(* Logix 5000 Program export KEP; software revision 30.00; part 13 of 15 *)
(* tags used below, declared in another part *)
   Ed25519_SIGN1 : Ed25519_SIGN;
   Ed25519_SIGN2 : Ed25519_SIGN;
   Ed25519_SIGN3 : Ed25519_SIGN;
   Ed25519_SIGN4 : Ed25519_SIGN;
   EdDSA_INTERNAL : EdDSA_INTERNAL[5];
   EdDSA_STATES : EdDSA_STATECTRL[15];
   InternalFlags : InternalFlags[5];
   InternalFlag_AllNodesUsingKsPrime : BOOL;
   InternalFlag_ALLOK : BOOL;
   InternalFlag_CreateNewKsPrime : BOOL;
   InternalFlag_KeyServerIdentityNo : BOOL;
   InternalFlag_KeyServerIdentityYes : BOOL;
   InternalFlag_KsEqualKsPrimeStatus : BOOL;
   InternalFlag_KsIDMatchesServer : BOOL;
   InternalFlag_KsPrimeAvail : BOOL;
   InternalFlag_KsPrimeIDMatchesServer : BOOL;
   InternalFlag_PowerOnCycle : BOOL;
   Internal_EdDSA_Msg : EdDSA_MSG;
   Internal_PriKeyPrefix : STRING;
   Internal_PriKeyScalar : STRING;
   Internal_PubKey : STRING;
   MyNodeNumber : DINT;
   ServerNode : INT;
   SignedMsgDest : INT;   // 0=None 1=Server 2=Client 3=All
   Temp_Processor_C1 : DINT[22];
   Temp_Processor_C10 : DINT[22];
   Temp_Processor_C2 : DINT[22];
   Temp_Processor_C3 : DINT[22];
   Temp_Processor_C4 : DINT[22];
   Temp_Processor_C5 : DINT[22];
   Temp_Processor_C6 : DINT[22];
   Temp_Processor_C7 : DINT[22];
   Temp_Processor_C8 : DINT[22];
   Temp_Processor_C9 : DINT[22];
   Temp_Processor_D1 : DINT[43];
   Temp_Processor_D2 : DINT[43];
   Temp_Processor_E1 : DINT[32];
   Temp_Processor_E2 : DINT[32];
   Temp_Processor_E3 : DINT[32];
   Temp_Processor_HASH : LINT[8];
   Temp_Processor_L : LINT[4];
   Temp_Processor_MSG : LINT[1600];
   Temp_Processor_P1 : POINT;
   Temp_Processor_P2 : POINT;
   Temp_Processor_P3 : POINT;
   Temp_Processor_P4 : POINT;
   Temp_Processor_S : STRING;
   T_INT1 : INT;
   WorkingNode : DINT;
   EdDSA_MSG_TO_NODE1 : EdDSA_MSG;
   EdDSA_MSG_TO_NODE2 : EdDSA_MSG;
   EdDSA_MSG_TO_NODE3 : EdDSA_MSG;
   EdDSA_MSG_TO_NODE4 : EdDSA_MSG;
   InternalFlag_KsID : LINT;
   InternalFlag_KsPrimeID : LINT;
   NODE : VMAC_DATA_INTERNAL[5];
(* KEP, continued *)

ROUTINE PROCESSOR_STATE4   (* ladder *)
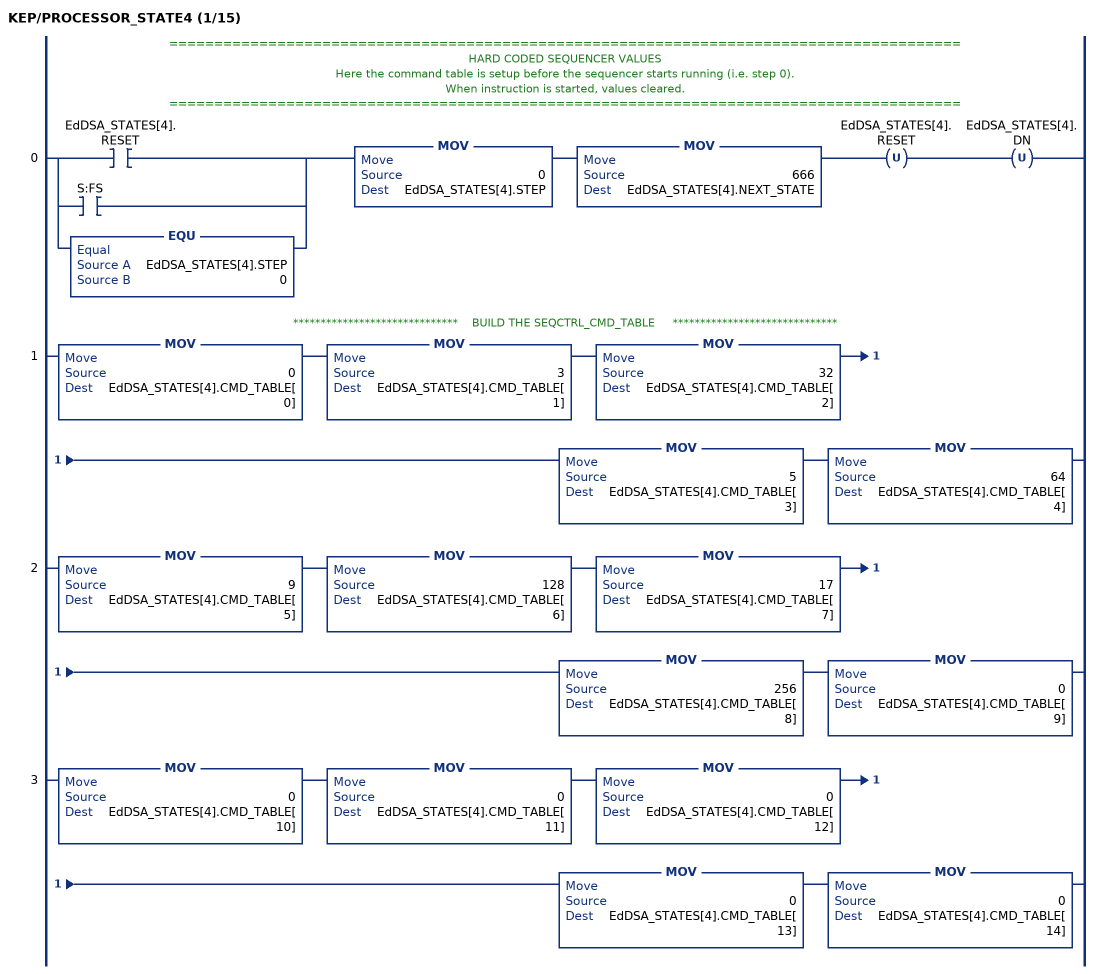
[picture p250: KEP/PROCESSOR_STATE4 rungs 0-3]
   // ========================================================================================
   // HARD CODED SEQUENCER VALUES
   // Here the command table is setup before the sequencer starts running (i.e. step 0).
   // When instruction is started, values cleared.
   // ========================================================================================
   0: [[XIC(EdDSA_STATES[4].RESET) ,XIC(S:FS) ] ,EQU(EdDSA_STATES[4].STEP,0) ]MOV(0,EdDSA_STATES[4].STEP)MOV(666,EdDSA_STATES[4].NEXT_STATE)OTU(EdDSA_STATES[4].RESET)OTU(EdDSA_STATES[4].DN);
   // ******************************    BUILD THE SEQCTRL_CMD_TABLE     ******************************
   1: MOV(0,EdDSA_STATES[4].CMD_TABLE[0])MOV(3,EdDSA_STATES[4].CMD_TABLE[1])MOV(32,EdDSA_STATES[4].CMD_TABLE[2])MOV(5,EdDSA_STATES[4].CMD_TABLE[3])MOV(64,EdDSA_STATES[4].CMD_TABLE[4]);
   2: MOV(9,EdDSA_STATES[4].CMD_TABLE[5])MOV(128,EdDSA_STATES[4].CMD_TABLE[6])MOV(17,EdDSA_STATES[4].CMD_TABLE[7])MOV(256,EdDSA_STATES[4].CMD_TABLE[8])MOV(0,EdDSA_STATES[4].CMD_TABLE[9]);
   3: MOV(0,EdDSA_STATES[4].CMD_TABLE[10])MOV(0,EdDSA_STATES[4].CMD_TABLE[11])MOV(0,EdDSA_STATES[4].CMD_TABLE[12])MOV(0,EdDSA_STATES[4].CMD_TABLE[13])MOV(0,EdDSA_STATES[4].CMD_TABLE[14]);
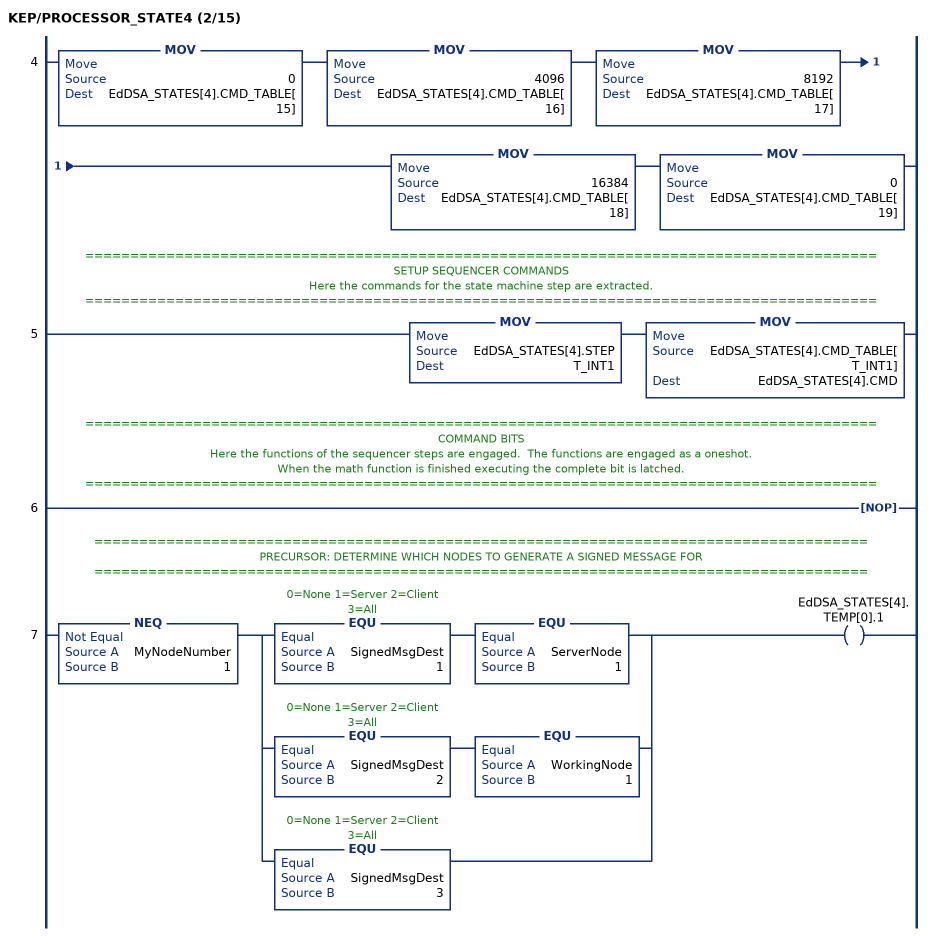
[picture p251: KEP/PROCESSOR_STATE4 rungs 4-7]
   4: MOV(0,EdDSA_STATES[4].CMD_TABLE[15])MOV(4096,EdDSA_STATES[4].CMD_TABLE[16])MOV(8192,EdDSA_STATES[4].CMD_TABLE[17])MOV(16384,EdDSA_STATES[4].CMD_TABLE[18])MOV(0,EdDSA_STATES[4].CMD_TABLE[19]);
   // ========================================================================================
   // SETUP SEQUENCER COMMANDS
   // Here the commands for the state machine step are extracted.
   // ========================================================================================
   5: MOV(EdDSA_STATES[4].STEP,T_INT1)MOV(EdDSA_STATES[4].CMD_TABLE[T_INT1],EdDSA_STATES[4].CMD);
   // ========================================================================================
   // COMMAND BITS
   // Here the functions of the sequencer steps are engaged.  The functions are engaged as a oneshot.
   // When the math function is finished executing the complete bit is latched.
   // ========================================================================================
   6: NOP();
   // ======================================================================================
   // PRECURSOR: DETERMINE WHICH NODES TO GENERATE A SIGNED MESSAGE FOR
   // ======================================================================================
   7: NEQ(MyNodeNumber,1)[EQU(SignedMsgDest,1) EQU(ServerNode,1) ,EQU(SignedMsgDest,2) EQU(WorkingNode,1) ,EQU(SignedMsgDest,3) ]OTE(EdDSA_STATES[4].TEMP[0].1);
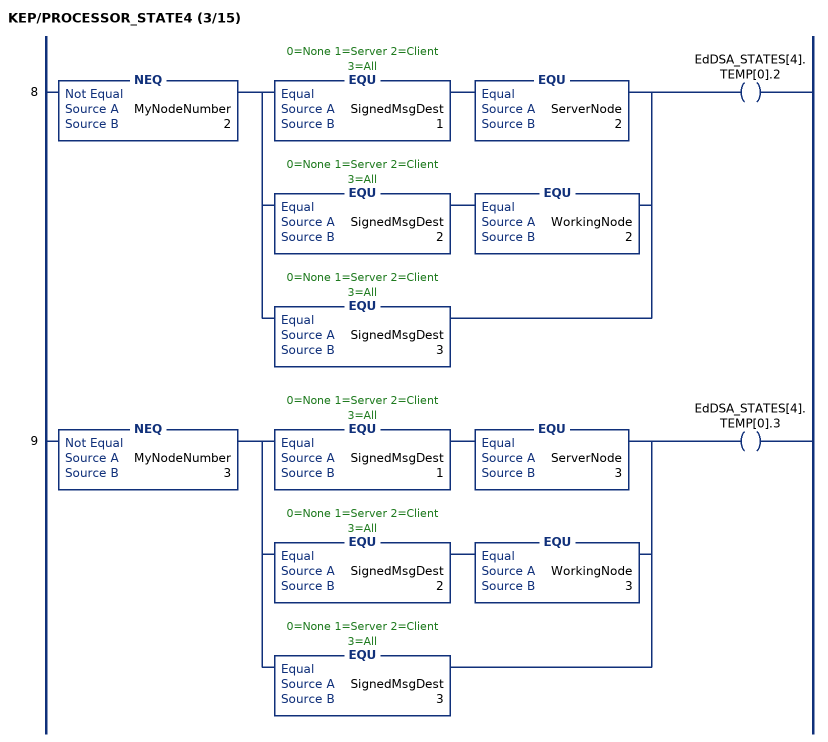
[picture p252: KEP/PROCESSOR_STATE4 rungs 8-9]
   8: NEQ(MyNodeNumber,2)[EQU(SignedMsgDest,1) EQU(ServerNode,2) ,EQU(SignedMsgDest,2) EQU(WorkingNode,2) ,EQU(SignedMsgDest,3) ]OTE(EdDSA_STATES[4].TEMP[0].2);
   9: NEQ(MyNodeNumber,3)[EQU(SignedMsgDest,1) EQU(ServerNode,3) ,EQU(SignedMsgDest,2) EQU(WorkingNode,3) ,EQU(SignedMsgDest,3) ]OTE(EdDSA_STATES[4].TEMP[0].3);
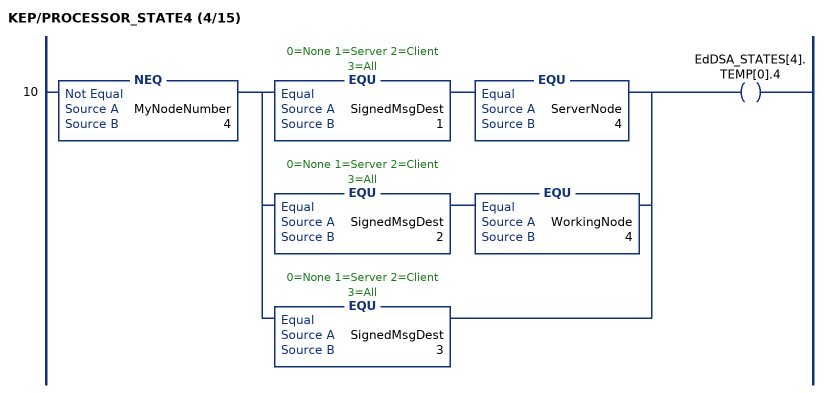
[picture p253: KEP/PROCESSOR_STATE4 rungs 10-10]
   10: NEQ(MyNodeNumber,4)[EQU(SignedMsgDest,1) EQU(ServerNode,4) ,EQU(SignedMsgDest,2) EQU(WorkingNode,4) ,EQU(SignedMsgDest,3) ]OTE(EdDSA_STATES[4].TEMP[0].4);
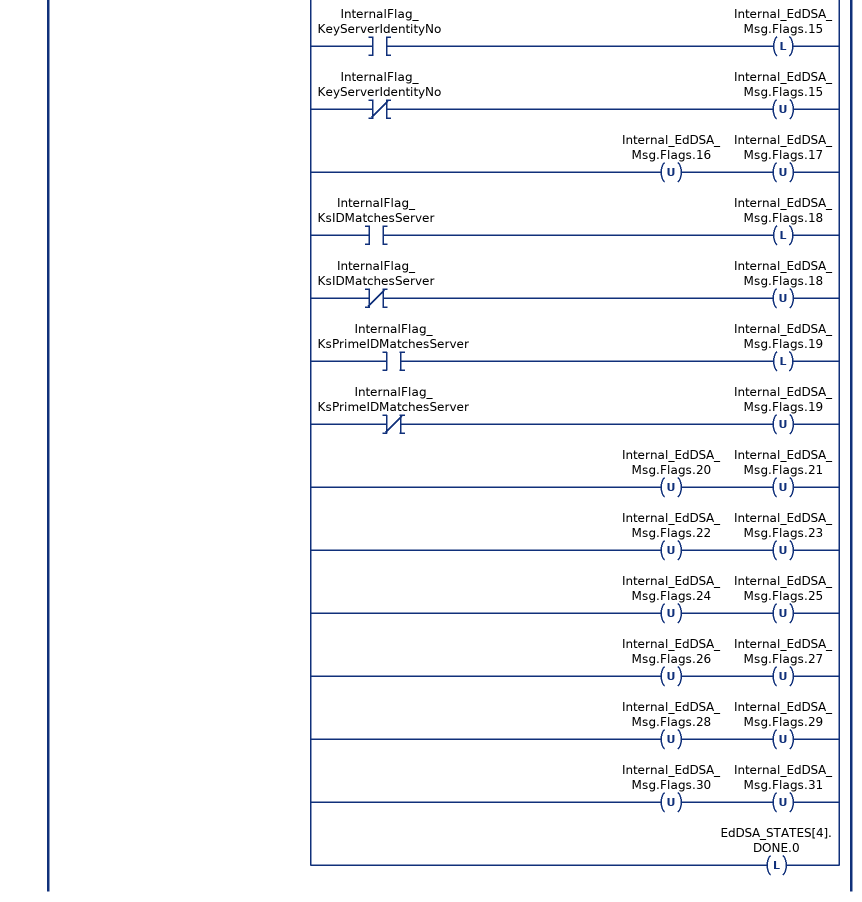
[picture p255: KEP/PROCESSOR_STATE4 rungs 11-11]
   // ======================================================================================
   // PART 0: MAP KEY IDENTITY AND COMMON FLAGS TO INTERNAL EdDSA MESSAGE
   // ======================================================================================
   11: XIC(EdDSA_STATES[4].CMD.0)XIO(EdDSA_STATES[4].DONE.0)[COP(InternalFlag_KsID,Internal_EdDSA_Msg.KsID,1) COP(InternalFlag_KsPrimeID,Internal_EdDSA_Msg.KsPrimeID,1) ,[XIC(InternalFlag_ALLOK) OTL(Internal_EdDSA_Msg.Flags.0) ,XIO(InternalFlag_ALLOK) OTU(Internal_EdDSA_Msg.Flags.0) ] ,OTU(Internal_EdDSA_Msg.Flags.1) OTU(Internal_EdDSA_Msg.Flags.2) ,OTU(Internal_EdDSA_Msg.Flags.3) OTU(Internal_EdDSA_Msg.Flags.4) ,OTU(Internal_EdDSA_Msg.Flags.5) OTU(Internal_EdDSA_Msg.Flags.6) ,[XIC(InternalFlag_KsPrimeAvail) OTL(Internal_EdDSA_Msg.Flags.9) ,XIO(InternalFlag_KsPrimeAvail) OTU(Internal_EdDSA_Msg.Flags.9) ] ,OTU(Internal_EdDSA_Msg.Flags.10) OTU(Internal_EdDSA_Msg.Flags.11) ,[XIC(InternalFlag_KsEqualKsPrimeStatus) OTL(Internal_EdDSA_Msg.Flags.12) ,XIO(InternalFlag_KsEqualKsPrimeStatus) OTU(Internal_EdDSA_Msg.Flags.12) ] ,OTU(Internal_EdDSA_Msg.Flags.13) ,[XIC(InternalFlag_KeyServerIdentityYes) OTL(Internal_EdDSA_Msg.Flags.14) ,XIO(InternalFlag_KeyServerIdentityYes) OTU(Internal_EdDSA_Msg.Flags.14) ] ,[XIC(InternalFlag_KeyServerIdentityNo) OTL(Internal_EdDSA_Msg.Flags.15) ,XIO(InternalFlag_KeyServerIdentityNo) OTU(Internal_EdDSA_Msg.Flags.15) ] ,OTU(Internal_EdDSA_Msg.Flags.16) OTU(Internal_EdDSA_Msg.Flags.17) ,[XIC(InternalFlag_KsIDMatchesServer) OTL(Internal_EdDSA_Msg.Flags.18) ,XIO(InternalFlag_KsIDMatchesServer) OTU(Internal_EdDSA_Msg.Flags.18) ] ,[XIC(InternalFlag_KsPrimeIDMatchesServer) OTL(Internal_EdDSA_Msg.Flags.19) ,XIO(InternalFlag_KsPrimeIDMatchesServer) OTU(Internal_EdDSA_Msg.Flags.19) ] ,OTU(Internal_EdDSA_Msg.Flags.20) OTU(Internal_EdDSA_Msg.Flags.21) ,OTU(Internal_EdDSA_Msg.Flags.22) OTU(Internal_EdDSA_Msg.Flags.23) ,OTU(Internal_EdDSA_Msg.Flags.24) OTU(Internal_EdDSA_Msg.Flags.25) ,OTU(Internal_EdDSA_Msg.Flags.26) OTU(Internal_EdDSA_Msg.Flags.27) ,OTU(Internal_EdDSA_Msg.Flags.28) OTU(Internal_EdDSA_Msg.Flags.29) ,OTU(Internal_EdDSA_Msg.Flags.30) OTU(Internal_EdDSA_Msg.Flags.31) ,OTL(EdDSA_STATES[4].DONE.0) ];
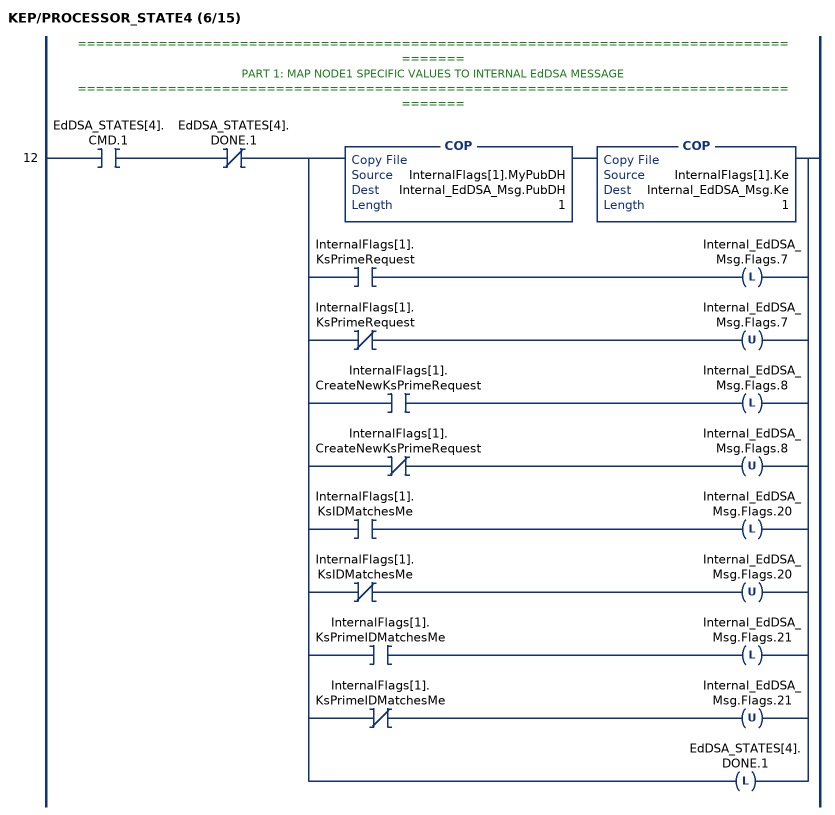
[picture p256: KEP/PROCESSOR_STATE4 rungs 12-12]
   // ======================================================================================
   // PART 1: MAP NODE1 SPECIFIC VALUES TO INTERNAL EdDSA MESSAGE
   // ======================================================================================
   12: XIC(EdDSA_STATES[4].CMD.1)XIO(EdDSA_STATES[4].DONE.1)[COP(InternalFlags[1].MyPubDH,Internal_EdDSA_Msg.PubDH,1) COP(InternalFlags[1].Ke,Internal_EdDSA_Msg.Ke,1) ,[XIC(InternalFlags[1].KsPrimeRequest) OTL(Internal_EdDSA_Msg.Flags.7) ,XIO(InternalFlags[1].KsPrimeRequest) OTU(Internal_EdDSA_Msg.Flags.7) ] ,[XIC(InternalFlags[1].CreateNewKsPrimeRequest) OTL(Internal_EdDSA_Msg.Flags.8) ,XIO(InternalFlags[1].CreateNewKsPrimeRequest) OTU(Internal_EdDSA_Msg.Flags.8) ] ,[XIC(InternalFlags[1].KsIDMatchesMe) OTL(Internal_EdDSA_Msg.Flags.20) ,XIO(InternalFlags[1].KsIDMatchesMe) OTU(Internal_EdDSA_Msg.Flags.20) ] ,[XIC(InternalFlags[1].KsPrimeIDMatchesMe) OTL(Internal_EdDSA_Msg.Flags.21) ,XIO(InternalFlags[1].KsPrimeIDMatchesMe) OTU(Internal_EdDSA_Msg.Flags.21) ] ,OTL(EdDSA_STATES[4].DONE.1) ];
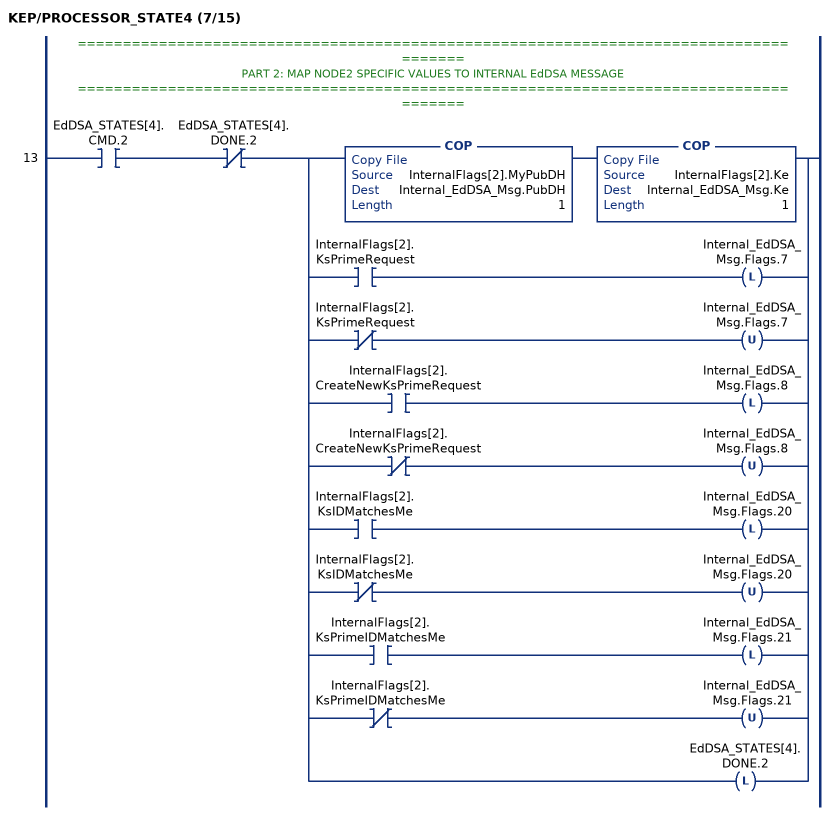
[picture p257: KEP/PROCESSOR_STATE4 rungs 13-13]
   // ======================================================================================
   // PART 2: MAP NODE2 SPECIFIC VALUES TO INTERNAL EdDSA MESSAGE
   // ======================================================================================
   13: XIC(EdDSA_STATES[4].CMD.2)XIO(EdDSA_STATES[4].DONE.2)[COP(InternalFlags[2].MyPubDH,Internal_EdDSA_Msg.PubDH,1) COP(InternalFlags[2].Ke,Internal_EdDSA_Msg.Ke,1) ,[XIC(InternalFlags[2].KsPrimeRequest) OTL(Internal_EdDSA_Msg.Flags.7) ,XIO(InternalFlags[2].KsPrimeRequest) OTU(Internal_EdDSA_Msg.Flags.7) ] ,[XIC(InternalFlags[2].CreateNewKsPrimeRequest) OTL(Internal_EdDSA_Msg.Flags.8) ,XIO(InternalFlags[2].CreateNewKsPrimeRequest) OTU(Internal_EdDSA_Msg.Flags.8) ] ,[XIC(InternalFlags[2].KsIDMatchesMe) OTL(Internal_EdDSA_Msg.Flags.20) ,XIO(InternalFlags[2].KsIDMatchesMe) OTU(Internal_EdDSA_Msg.Flags.20) ] ,[XIC(InternalFlags[2].KsPrimeIDMatchesMe) OTL(Internal_EdDSA_Msg.Flags.21) ,XIO(InternalFlags[2].KsPrimeIDMatchesMe) OTU(Internal_EdDSA_Msg.Flags.21) ] ,OTL(EdDSA_STATES[4].DONE.2) ];
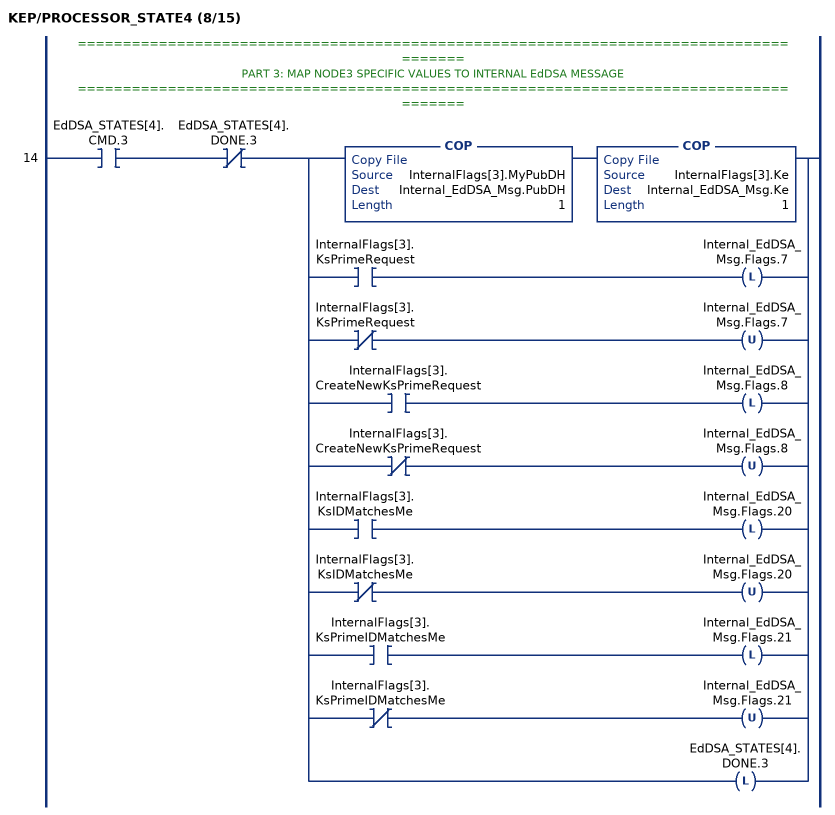
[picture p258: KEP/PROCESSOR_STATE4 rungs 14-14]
   // ======================================================================================
   // PART 3: MAP NODE3 SPECIFIC VALUES TO INTERNAL EdDSA MESSAGE
   // ======================================================================================
   14: XIC(EdDSA_STATES[4].CMD.3)XIO(EdDSA_STATES[4].DONE.3)[COP(InternalFlags[3].MyPubDH,Internal_EdDSA_Msg.PubDH,1) COP(InternalFlags[3].Ke,Internal_EdDSA_Msg.Ke,1) ,[XIC(InternalFlags[3].KsPrimeRequest) OTL(Internal_EdDSA_Msg.Flags.7) ,XIO(InternalFlags[3].KsPrimeRequest) OTU(Internal_EdDSA_Msg.Flags.7) ] ,[XIC(InternalFlags[3].CreateNewKsPrimeRequest) OTL(Internal_EdDSA_Msg.Flags.8) ,XIO(InternalFlags[3].CreateNewKsPrimeRequest) OTU(Internal_EdDSA_Msg.Flags.8) ] ,[XIC(InternalFlags[3].KsIDMatchesMe) OTL(Internal_EdDSA_Msg.Flags.20) ,XIO(InternalFlags[3].KsIDMatchesMe) OTU(Internal_EdDSA_Msg.Flags.20) ] ,[XIC(InternalFlags[3].KsPrimeIDMatchesMe) OTL(Internal_EdDSA_Msg.Flags.21) ,XIO(InternalFlags[3].KsPrimeIDMatchesMe) OTU(Internal_EdDSA_Msg.Flags.21) ] ,OTL(EdDSA_STATES[4].DONE.3) ];
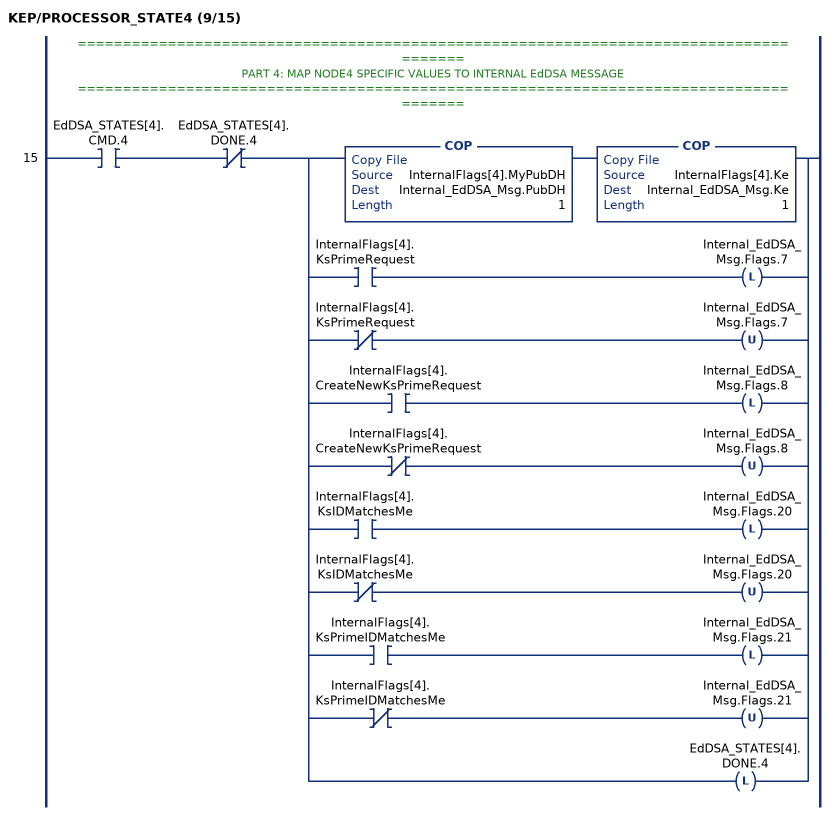
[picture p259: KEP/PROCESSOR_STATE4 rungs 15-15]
   // ======================================================================================
   // PART 4: MAP NODE4 SPECIFIC VALUES TO INTERNAL EdDSA MESSAGE
   // ======================================================================================
   15: XIC(EdDSA_STATES[4].CMD.4)XIO(EdDSA_STATES[4].DONE.4)[COP(InternalFlags[4].MyPubDH,Internal_EdDSA_Msg.PubDH,1) COP(InternalFlags[4].Ke,Internal_EdDSA_Msg.Ke,1) ,[XIC(InternalFlags[4].KsPrimeRequest) OTL(Internal_EdDSA_Msg.Flags.7) ,XIO(InternalFlags[4].KsPrimeRequest) OTU(Internal_EdDSA_Msg.Flags.7) ] ,[XIC(InternalFlags[4].CreateNewKsPrimeRequest) OTL(Internal_EdDSA_Msg.Flags.8) ,XIO(InternalFlags[4].CreateNewKsPrimeRequest) OTU(Internal_EdDSA_Msg.Flags.8) ] ,[XIC(InternalFlags[4].KsIDMatchesMe) OTL(Internal_EdDSA_Msg.Flags.20) ,XIO(InternalFlags[4].KsIDMatchesMe) OTU(Internal_EdDSA_Msg.Flags.20) ] ,[XIC(InternalFlags[4].KsPrimeIDMatchesMe) OTL(Internal_EdDSA_Msg.Flags.21) ,XIO(InternalFlags[4].KsPrimeIDMatchesMe) OTU(Internal_EdDSA_Msg.Flags.21) ] ,OTL(EdDSA_STATES[4].DONE.4) ];
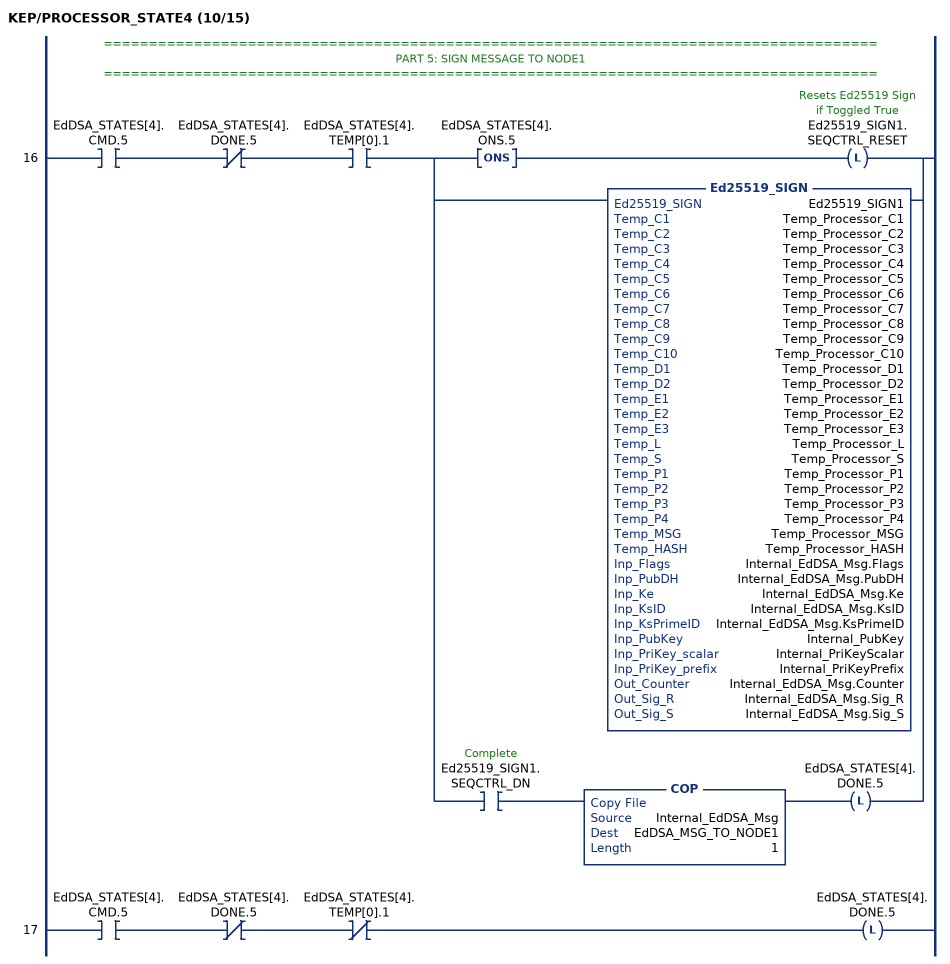
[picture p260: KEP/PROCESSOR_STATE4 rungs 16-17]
   // ======================================================================================
   // PART 5: SIGN MESSAGE TO NODE1
   // ======================================================================================
   16: XIC(EdDSA_STATES[4].CMD.5)XIO(EdDSA_STATES[4].DONE.5)XIC(EdDSA_STATES[4].TEMP[0].1)[ONS(EdDSA_STATES[4].ONS.5) OTL(Ed25519_SIGN1.SEQCTRL_RESET) ,Ed25519_SIGN(Ed25519_SIGN1,Temp_Processor_C1,Temp_Processor_C2,Temp_Processor_C3,Temp_Processor_C4,Temp_Processor_C5,Temp_Processor_C6,Temp_Processor_C7,Temp_Processor_C8,Temp_Processor_C9,Temp_Processor_C10,Temp_Processor_D1,Temp_Processor_D2,Temp_Processor_E1,Temp_Processor_E2,Temp_Processor_E3,Temp_Processor_L,Temp_Processor_S,Temp_Processor_P1,Temp_Processor_P2,Temp_Processor_P3,Temp_Processor_P4,Temp_Processor_MSG,Temp_Processor_HASH,Internal_EdDSA_Msg.Flags,Internal_EdDSA_Msg.PubDH,Internal_EdDSA_Msg.Ke,Internal_EdDSA_Msg.KsID,Internal_EdDSA_Msg.KsPrimeID,Internal_PubKey,Internal_PriKeyScalar,Internal_PriKeyPrefix,Internal_EdDSA_Msg.Counter,Internal_EdDSA_Msg.Sig_R,Internal_EdDSA_Msg.Sig_S) ,XIC(Ed25519_SIGN1.SEQCTRL_DN) COP(Internal_EdDSA_Msg,EdDSA_MSG_TO_NODE1,1) OTL(EdDSA_STATES[4].DONE.5) ];
   17: XIC(EdDSA_STATES[4].CMD.5)XIO(EdDSA_STATES[4].DONE.5)XIO(EdDSA_STATES[4].TEMP[0].1)OTL(EdDSA_STATES[4].DONE.5);
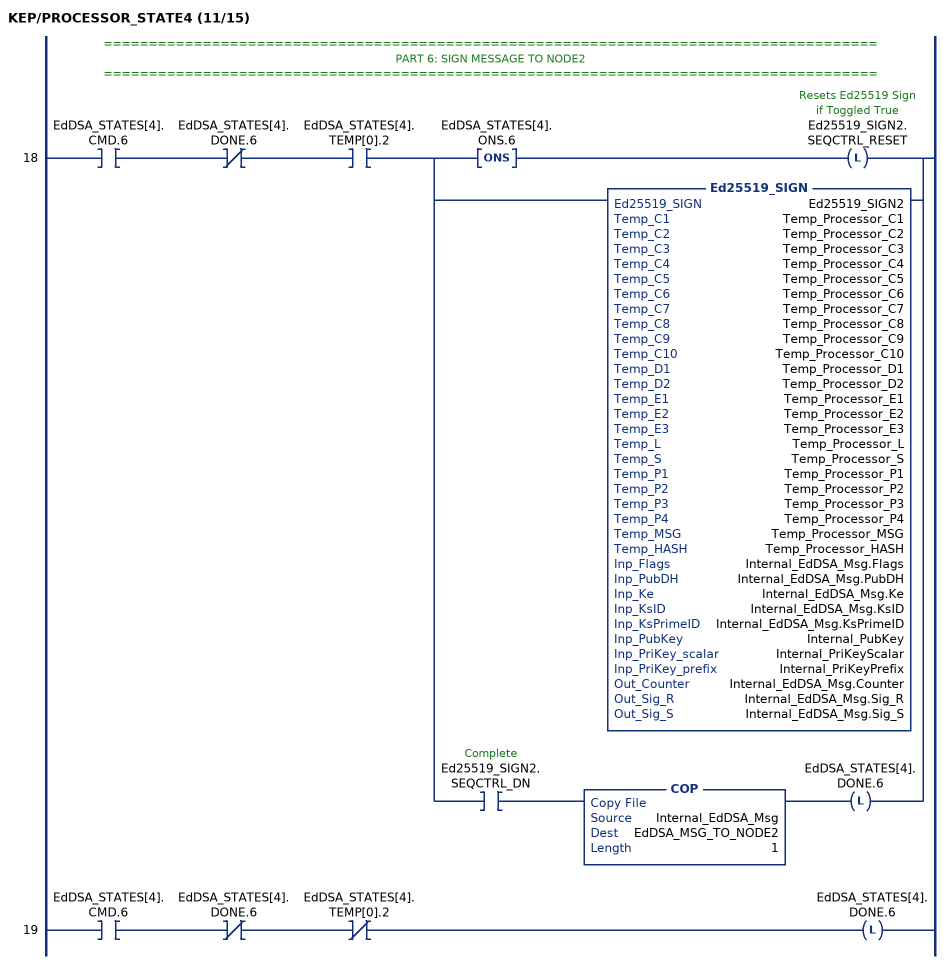
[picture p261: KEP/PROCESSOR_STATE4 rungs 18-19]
   // ======================================================================================
   // PART 6: SIGN MESSAGE TO NODE2
   // ======================================================================================
   18: XIC(EdDSA_STATES[4].CMD.6)XIO(EdDSA_STATES[4].DONE.6)XIC(EdDSA_STATES[4].TEMP[0].2)[ONS(EdDSA_STATES[4].ONS.6) OTL(Ed25519_SIGN2.SEQCTRL_RESET) ,Ed25519_SIGN(Ed25519_SIGN2,Temp_Processor_C1,Temp_Processor_C2,Temp_Processor_C3,Temp_Processor_C4,Temp_Processor_C5,Temp_Processor_C6,Temp_Processor_C7,Temp_Processor_C8,Temp_Processor_C9,Temp_Processor_C10,Temp_Processor_D1,Temp_Processor_D2,Temp_Processor_E1,Temp_Processor_E2,Temp_Processor_E3,Temp_Processor_L,Temp_Processor_S,Temp_Processor_P1,Temp_Processor_P2,Temp_Processor_P3,Temp_Processor_P4,Temp_Processor_MSG,Temp_Processor_HASH,Internal_EdDSA_Msg.Flags,Internal_EdDSA_Msg.PubDH,Internal_EdDSA_Msg.Ke,Internal_EdDSA_Msg.KsID,Internal_EdDSA_Msg.KsPrimeID,Internal_PubKey,Internal_PriKeyScalar,Internal_PriKeyPrefix,Internal_EdDSA_Msg.Counter,Internal_EdDSA_Msg.Sig_R,Internal_EdDSA_Msg.Sig_S) ,XIC(Ed25519_SIGN2.SEQCTRL_DN) COP(Internal_EdDSA_Msg,EdDSA_MSG_TO_NODE2,1) OTL(EdDSA_STATES[4].DONE.6) ];
   19: XIC(EdDSA_STATES[4].CMD.6)XIO(EdDSA_STATES[4].DONE.6)XIO(EdDSA_STATES[4].TEMP[0].2)OTL(EdDSA_STATES[4].DONE.6);
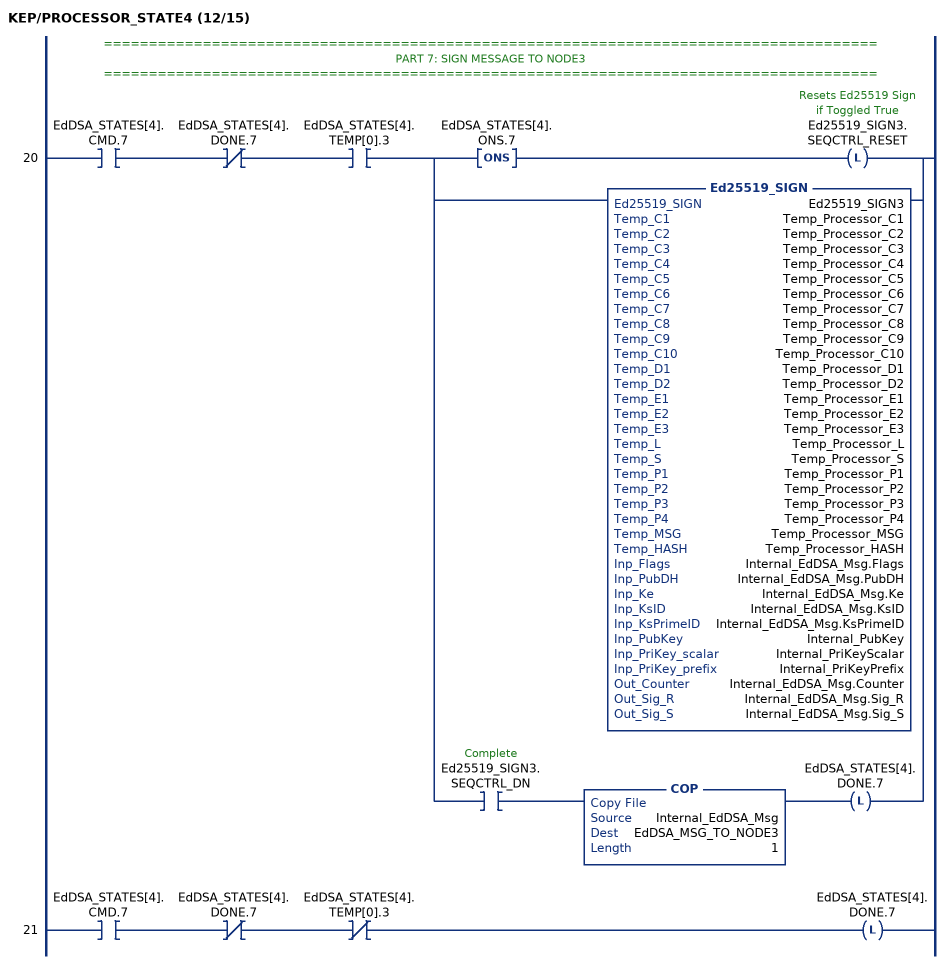
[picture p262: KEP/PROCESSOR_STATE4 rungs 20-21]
   // ======================================================================================
   // PART 7: SIGN MESSAGE TO NODE3
   // ======================================================================================
   20: XIC(EdDSA_STATES[4].CMD.7)XIO(EdDSA_STATES[4].DONE.7)XIC(EdDSA_STATES[4].TEMP[0].3)[ONS(EdDSA_STATES[4].ONS.7) OTL(Ed25519_SIGN3.SEQCTRL_RESET) ,Ed25519_SIGN(Ed25519_SIGN3,Temp_Processor_C1,Temp_Processor_C2,Temp_Processor_C3,Temp_Processor_C4,Temp_Processor_C5,Temp_Processor_C6,Temp_Processor_C7,Temp_Processor_C8,Temp_Processor_C9,Temp_Processor_C10,Temp_Processor_D1,Temp_Processor_D2,Temp_Processor_E1,Temp_Processor_E2,Temp_Processor_E3,Temp_Processor_L,Temp_Processor_S,Temp_Processor_P1,Temp_Processor_P2,Temp_Processor_P3,Temp_Processor_P4,Temp_Processor_MSG,Temp_Processor_HASH,Internal_EdDSA_Msg.Flags,Internal_EdDSA_Msg.PubDH,Internal_EdDSA_Msg.Ke,Internal_EdDSA_Msg.KsID,Internal_EdDSA_Msg.KsPrimeID,Internal_PubKey,Internal_PriKeyScalar,Internal_PriKeyPrefix,Internal_EdDSA_Msg.Counter,Internal_EdDSA_Msg.Sig_R,Internal_EdDSA_Msg.Sig_S) ,XIC(Ed25519_SIGN3.SEQCTRL_DN) COP(Internal_EdDSA_Msg,EdDSA_MSG_TO_NODE3,1) OTL(EdDSA_STATES[4].DONE.7) ];
   21: XIC(EdDSA_STATES[4].CMD.7)XIO(EdDSA_STATES[4].DONE.7)XIO(EdDSA_STATES[4].TEMP[0].3)OTL(EdDSA_STATES[4].DONE.7);
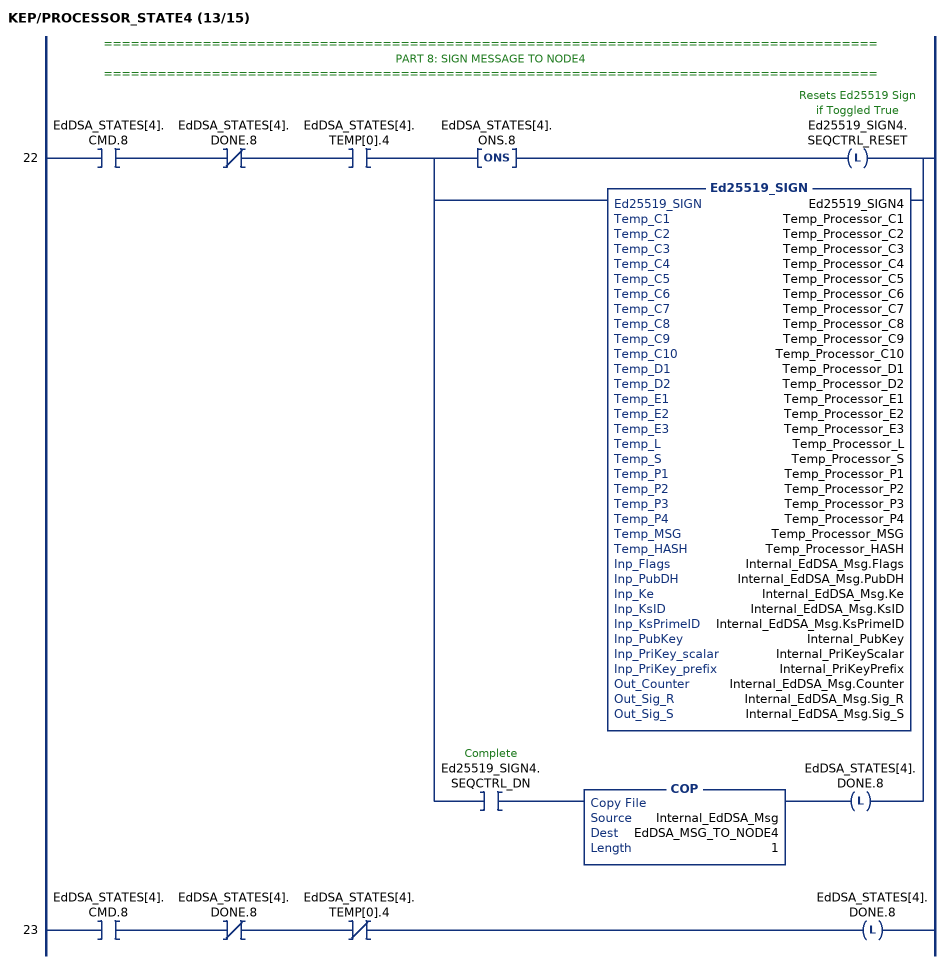
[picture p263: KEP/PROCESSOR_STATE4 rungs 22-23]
   // ======================================================================================
   // PART 8: SIGN MESSAGE TO NODE4
   // ======================================================================================
   22: XIC(EdDSA_STATES[4].CMD.8)XIO(EdDSA_STATES[4].DONE.8)XIC(EdDSA_STATES[4].TEMP[0].4)[ONS(EdDSA_STATES[4].ONS.8) OTL(Ed25519_SIGN4.SEQCTRL_RESET) ,Ed25519_SIGN(Ed25519_SIGN4,Temp_Processor_C1,Temp_Processor_C2,Temp_Processor_C3,Temp_Processor_C4,Temp_Processor_C5,Temp_Processor_C6,Temp_Processor_C7,Temp_Processor_C8,Temp_Processor_C9,Temp_Processor_C10,Temp_Processor_D1,Temp_Processor_D2,Temp_Processor_E1,Temp_Processor_E2,Temp_Processor_E3,Temp_Processor_L,Temp_Processor_S,Temp_Processor_P1,Temp_Processor_P2,Temp_Processor_P3,Temp_Processor_P4,Temp_Processor_MSG,Temp_Processor_HASH,Internal_EdDSA_Msg.Flags,Internal_EdDSA_Msg.PubDH,Internal_EdDSA_Msg.Ke,Internal_EdDSA_Msg.KsID,Internal_EdDSA_Msg.KsPrimeID,Internal_PubKey,Internal_PriKeyScalar,Internal_PriKeyPrefix,Internal_EdDSA_Msg.Counter,Internal_EdDSA_Msg.Sig_R,Internal_EdDSA_Msg.Sig_S) ,XIC(Ed25519_SIGN4.SEQCTRL_DN) COP(Internal_EdDSA_Msg,EdDSA_MSG_TO_NODE4,1) OTL(EdDSA_STATES[4].DONE.8) ];
   23: XIC(EdDSA_STATES[4].CMD.8)XIO(EdDSA_STATES[4].DONE.8)XIO(EdDSA_STATES[4].TEMP[0].4)OTL(EdDSA_STATES[4].DONE.8);
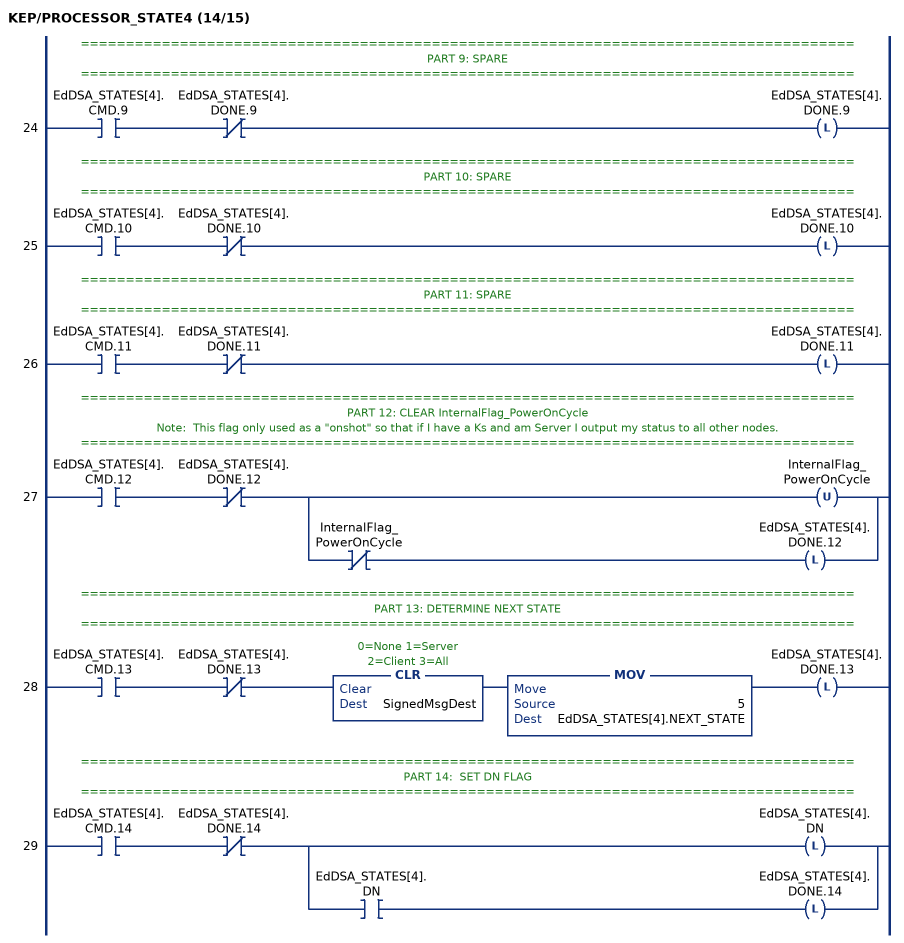
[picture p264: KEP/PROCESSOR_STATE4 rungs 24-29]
   // ======================================================================================
   // PART 9: SPARE
   // ======================================================================================
   24: XIC(EdDSA_STATES[4].CMD.9)XIO(EdDSA_STATES[4].DONE.9)OTL(EdDSA_STATES[4].DONE.9);
   // ======================================================================================
   // PART 10: SPARE
   // ======================================================================================
   25: XIC(EdDSA_STATES[4].CMD.10)XIO(EdDSA_STATES[4].DONE.10)OTL(EdDSA_STATES[4].DONE.10);
   // ======================================================================================
   // PART 11: SPARE
   // ======================================================================================
   26: XIC(EdDSA_STATES[4].CMD.11)XIO(EdDSA_STATES[4].DONE.11)OTL(EdDSA_STATES[4].DONE.11);
   // ======================================================================================
   // PART 12: CLEAR InternalFlag_PowerOnCycle
   // Note:  This flag only used as a "onshot" so that if I have a Ks and am Server I output my status to all other nodes.
   // ======================================================================================
   27: XIC(EdDSA_STATES[4].CMD.12)XIO(EdDSA_STATES[4].DONE.12)[OTU(InternalFlag_PowerOnCycle) ,XIO(InternalFlag_PowerOnCycle) OTL(EdDSA_STATES[4].DONE.12) ];
   // ======================================================================================
   // PART 13: DETERMINE NEXT STATE
   // ======================================================================================
   28: XIC(EdDSA_STATES[4].CMD.13)XIO(EdDSA_STATES[4].DONE.13)CLR(SignedMsgDest)MOV(5,EdDSA_STATES[4].NEXT_STATE)OTL(EdDSA_STATES[4].DONE.13);
   // ======================================================================================
   // PART 14:  SET DN FLAG
   // ======================================================================================
   29: XIC(EdDSA_STATES[4].CMD.14)XIO(EdDSA_STATES[4].DONE.14)[OTL(EdDSA_STATES[4].DN) ,XIC(EdDSA_STATES[4].DN) OTL(EdDSA_STATES[4].DONE.14) ];
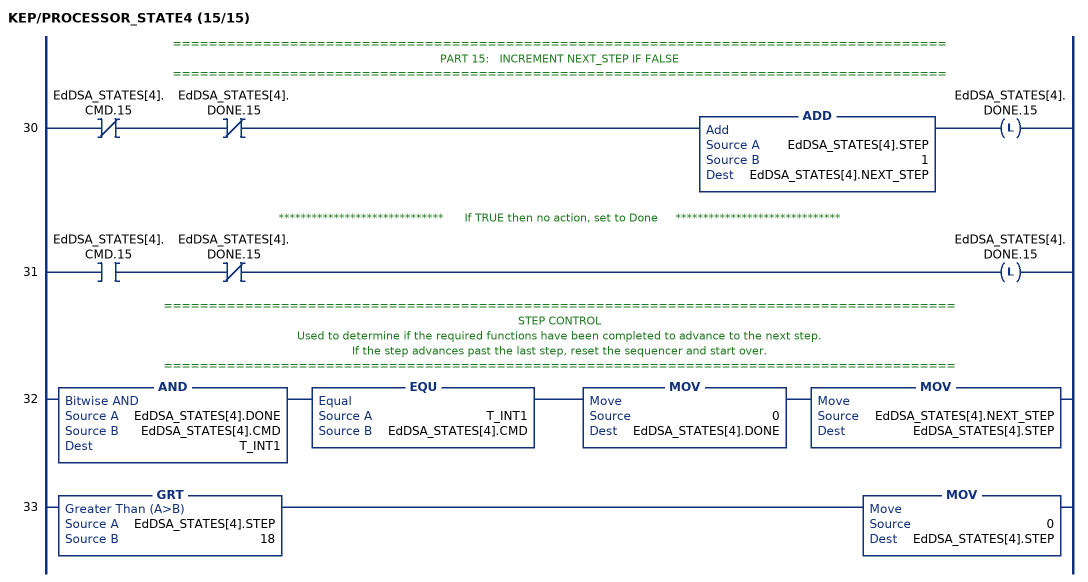
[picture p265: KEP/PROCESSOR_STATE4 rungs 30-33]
   // ======================================================================================
   // PART 15:   INCREMENT NEXT_STEP IF FALSE
   // ======================================================================================
   30: XIO(EdDSA_STATES[4].CMD.15)XIO(EdDSA_STATES[4].DONE.15)ADD(EdDSA_STATES[4].STEP,1,EdDSA_STATES[4].NEXT_STEP)OTL(EdDSA_STATES[4].DONE.15);
   // ******************************      If TRUE then no action, set to Done     ******************************
   31: XIC(EdDSA_STATES[4].CMD.15)XIO(EdDSA_STATES[4].DONE.15)OTL(EdDSA_STATES[4].DONE.15);
   // ========================================================================================
   // STEP CONTROL
   // Used to determine if the required functions have been completed to advance to the next step.
   // If the step advances past the last step, reset the sequencer and start over.
   // ========================================================================================
   32: AND(EdDSA_STATES[4].DONE,EdDSA_STATES[4].CMD,T_INT1)EQU(T_INT1,EdDSA_STATES[4].CMD)MOV(0,EdDSA_STATES[4].DONE)MOV(EdDSA_STATES[4].NEXT_STEP,EdDSA_STATES[4].STEP);
   33: GRT(EdDSA_STATES[4].STEP,18)MOV(0,EdDSA_STATES[4].STEP);
END_ROUTINE

ROUTINE PROCESSOR_STATE5   (* ladder *)
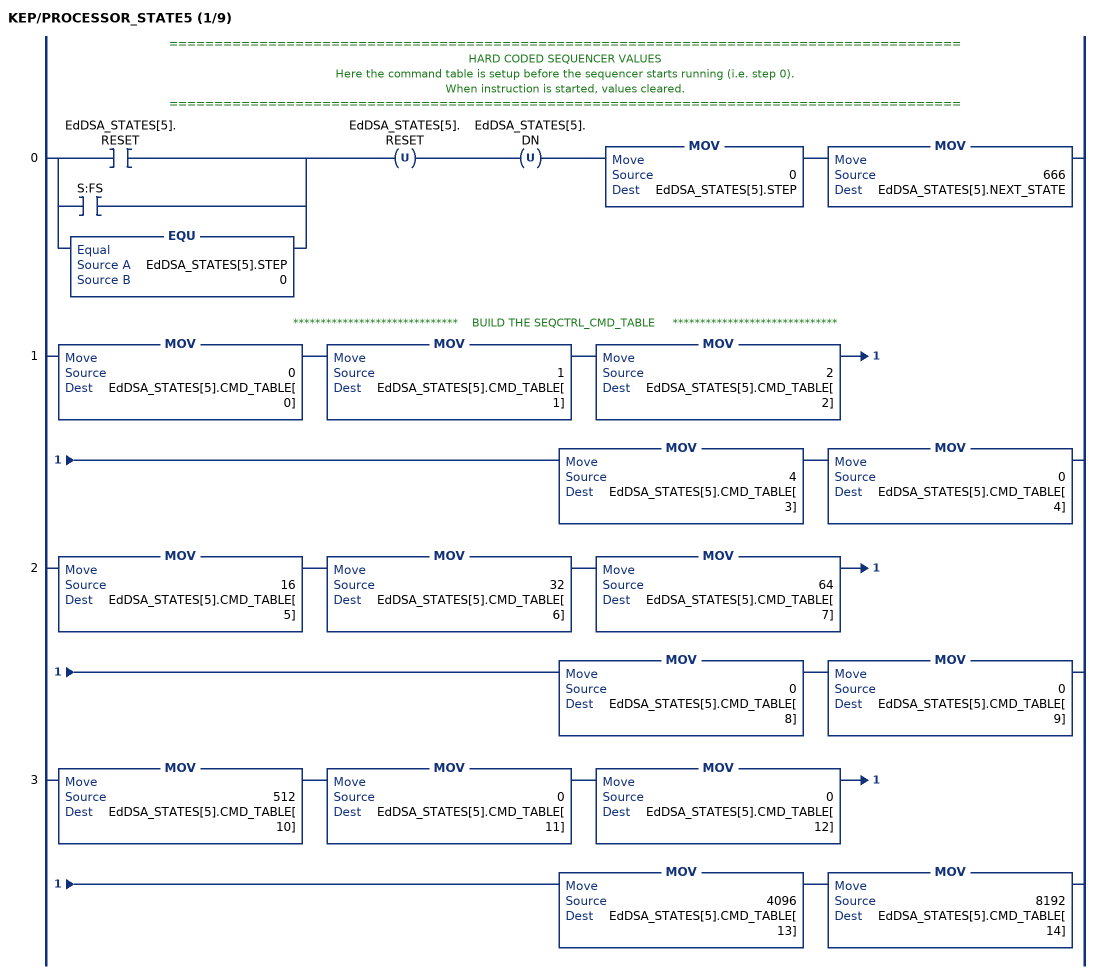
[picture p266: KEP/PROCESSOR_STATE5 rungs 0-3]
   // ========================================================================================
   // HARD CODED SEQUENCER VALUES
   // Here the command table is setup before the sequencer starts running (i.e. step 0).
   // When instruction is started, values cleared.
   // ========================================================================================
   0: [[XIC(EdDSA_STATES[5].RESET) ,XIC(S:FS) ] ,EQU(EdDSA_STATES[5].STEP,0) ]OTU(EdDSA_STATES[5].RESET)OTU(EdDSA_STATES[5].DN)MOV(0,EdDSA_STATES[5].STEP)MOV(666,EdDSA_STATES[5].NEXT_STATE);
   // ******************************    BUILD THE SEQCTRL_CMD_TABLE     ******************************
   1: MOV(0,EdDSA_STATES[5].CMD_TABLE[0])MOV(1,EdDSA_STATES[5].CMD_TABLE[1])MOV(2,EdDSA_STATES[5].CMD_TABLE[2])MOV(4,EdDSA_STATES[5].CMD_TABLE[3])MOV(0,EdDSA_STATES[5].CMD_TABLE[4]);
   2: MOV(16,EdDSA_STATES[5].CMD_TABLE[5])MOV(32,EdDSA_STATES[5].CMD_TABLE[6])MOV(64,EdDSA_STATES[5].CMD_TABLE[7])MOV(0,EdDSA_STATES[5].CMD_TABLE[8])MOV(0,EdDSA_STATES[5].CMD_TABLE[9]);
   3: MOV(512,EdDSA_STATES[5].CMD_TABLE[10])MOV(0,EdDSA_STATES[5].CMD_TABLE[11])MOV(0,EdDSA_STATES[5].CMD_TABLE[12])MOV(4096,EdDSA_STATES[5].CMD_TABLE[13])MOV(8192,EdDSA_STATES[5].CMD_TABLE[14]);
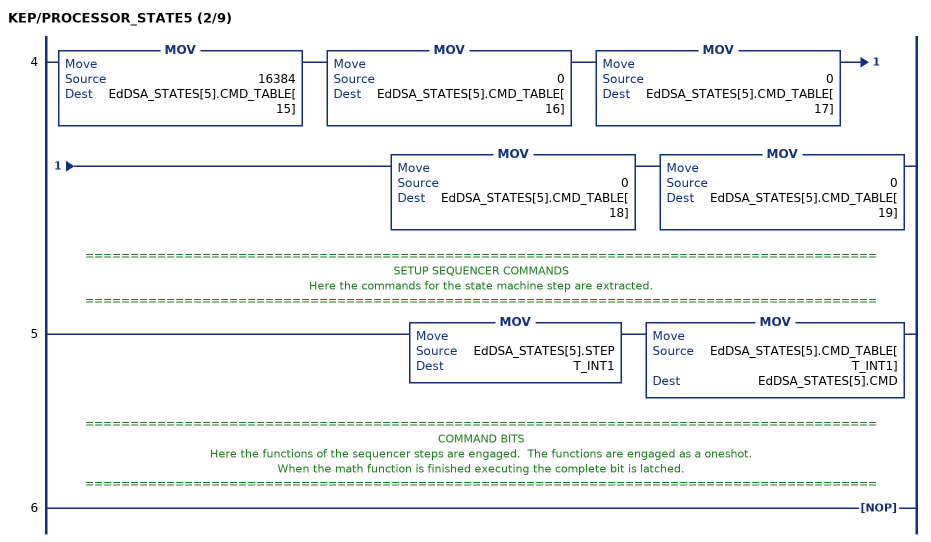
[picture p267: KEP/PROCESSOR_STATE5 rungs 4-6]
   4: MOV(16384,EdDSA_STATES[5].CMD_TABLE[15])MOV(0,EdDSA_STATES[5].CMD_TABLE[16])MOV(0,EdDSA_STATES[5].CMD_TABLE[17])MOV(0,EdDSA_STATES[5].CMD_TABLE[18])MOV(0,EdDSA_STATES[5].CMD_TABLE[19]);
   // ========================================================================================
   // SETUP SEQUENCER COMMANDS
   // Here the commands for the state machine step are extracted.
   // ========================================================================================
   5: MOV(EdDSA_STATES[5].STEP,T_INT1)MOV(EdDSA_STATES[5].CMD_TABLE[T_INT1],EdDSA_STATES[5].CMD);
   // ========================================================================================
   // COMMAND BITS
   // Here the functions of the sequencer steps are engaged.  The functions are engaged as a oneshot.
   // When the math function is finished executing the complete bit is latched.
   // ========================================================================================
   6: NOP();
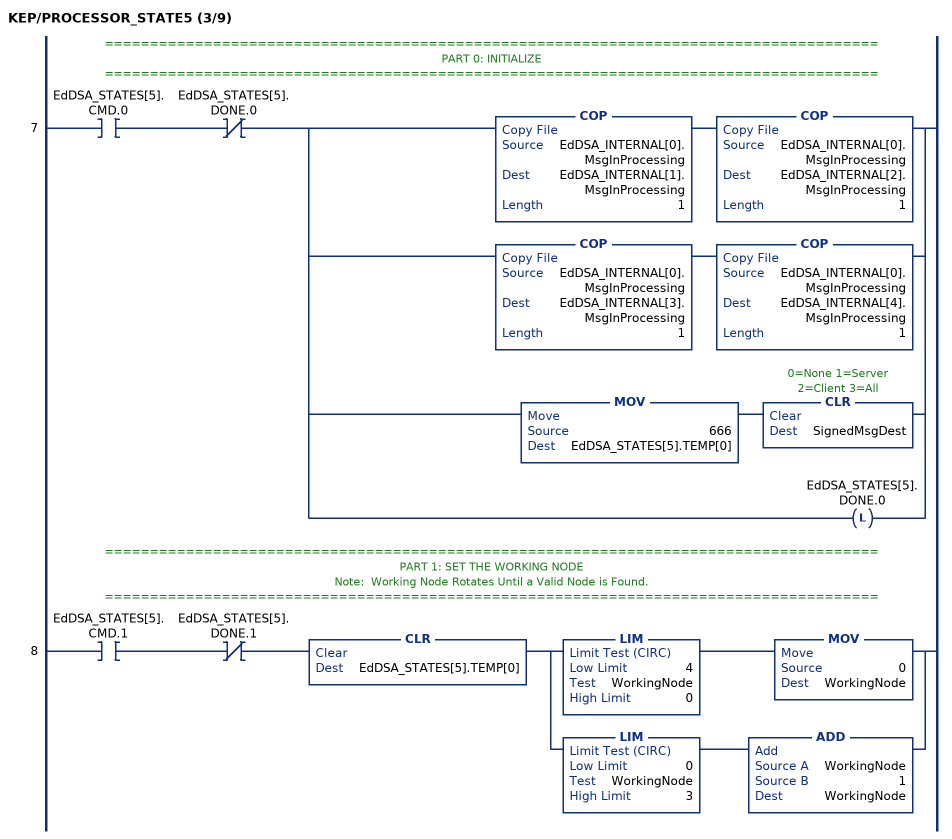
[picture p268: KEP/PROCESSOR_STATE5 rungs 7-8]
   // ======================================================================================
   // PART 0: INITIALIZE
   // ======================================================================================
   7: XIC(EdDSA_STATES[5].CMD.0)XIO(EdDSA_STATES[5].DONE.0)[COP(EdDSA_INTERNAL[0].MsgInProcessing,EdDSA_INTERNAL[1].MsgInProcessing,1) COP(EdDSA_INTERNAL[0].MsgInProcessing,EdDSA_INTERNAL[2].MsgInProcessing,1) ,COP(EdDSA_INTERNAL[0].MsgInProcessing,EdDSA_INTERNAL[3].MsgInProcessing,1) COP(EdDSA_INTERNAL[0].MsgInProcessing,EdDSA_INTERNAL[4].MsgInProcessing,1) ,MOV(666,EdDSA_STATES[5].TEMP[0]) CLR(SignedMsgDest) ,OTL(EdDSA_STATES[5].DONE.0) ];
   // ======================================================================================
   // PART 1: SET THE WORKING NODE
   // Note:  Working Node Rotates Until a Valid Node is Found.
   // ======================================================================================
   8: XIC(EdDSA_STATES[5].CMD.1)XIO(EdDSA_STATES[5].DONE.1)CLR(EdDSA_STATES[5].TEMP[0])[LIM(4,WorkingNode,0) MOV(0,WorkingNode) ,LIM(0,WorkingNode,3) ADD(WorkingNode,1,WorkingNode) ];
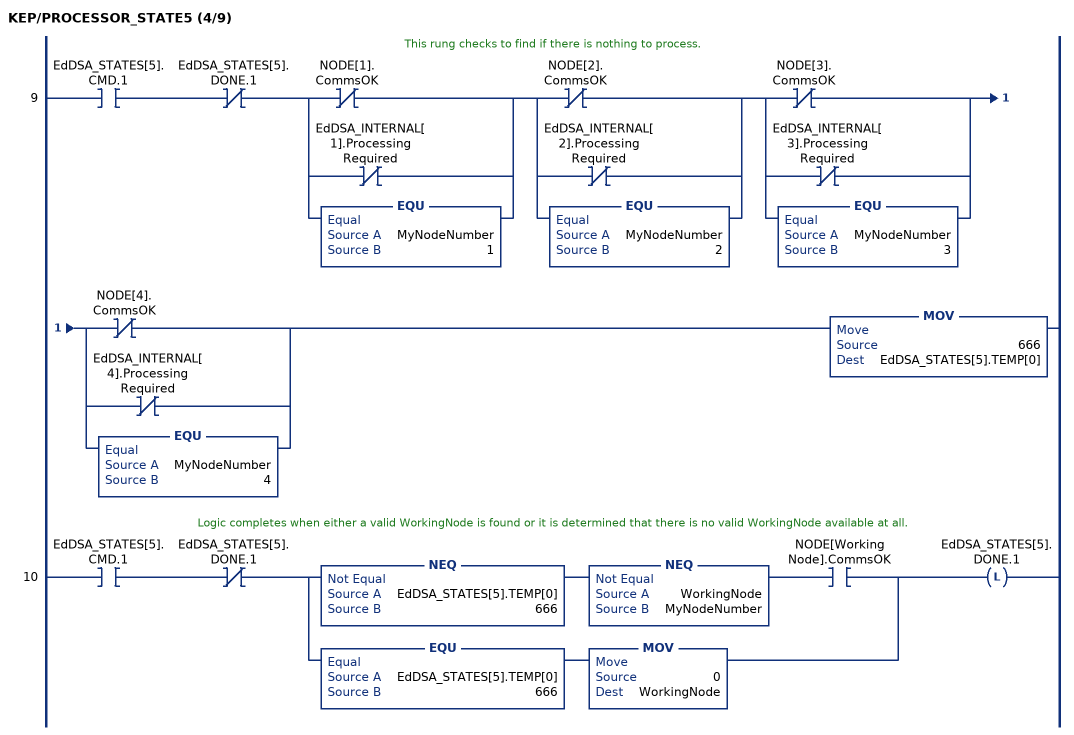
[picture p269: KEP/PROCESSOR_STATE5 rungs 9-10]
   // This rung checks to find if there is nothing to process.
   9: XIC(EdDSA_STATES[5].CMD.1)XIO(EdDSA_STATES[5].DONE.1)[XIO(NODE[1].CommsOK) ,XIO(EdDSA_INTERNAL[1].ProcessingRequired) ,EQU(MyNodeNumber,1) ][XIO(NODE[2].CommsOK) ,XIO(EdDSA_INTERNAL[2].ProcessingRequired) ,EQU(MyNodeNumber,2) ][XIO(NODE[3].CommsOK) ,XIO(EdDSA_INTERNAL[3].ProcessingRequired) ,EQU(MyNodeNumber,3) ][XIO(NODE[4].CommsOK) ,XIO(EdDSA_INTERNAL[4].ProcessingRequired) ,EQU(MyNodeNumber,4) ]MOV(666,EdDSA_STATES[5].TEMP[0]);
   // Logic completes when either a valid WorkingNode is found or it is determined that there is no valid WorkingNode available at all.
   10: XIC(EdDSA_STATES[5].CMD.1)XIO(EdDSA_STATES[5].DONE.1)[NEQ(EdDSA_STATES[5].TEMP[0],666) NEQ(WorkingNode,MyNodeNumber) XIC(NODE[WorkingNode].CommsOK) ,EQU(EdDSA_STATES[5].TEMP[0],666) MOV(0,WorkingNode) ]OTL(EdDSA_STATES[5].DONE.1);
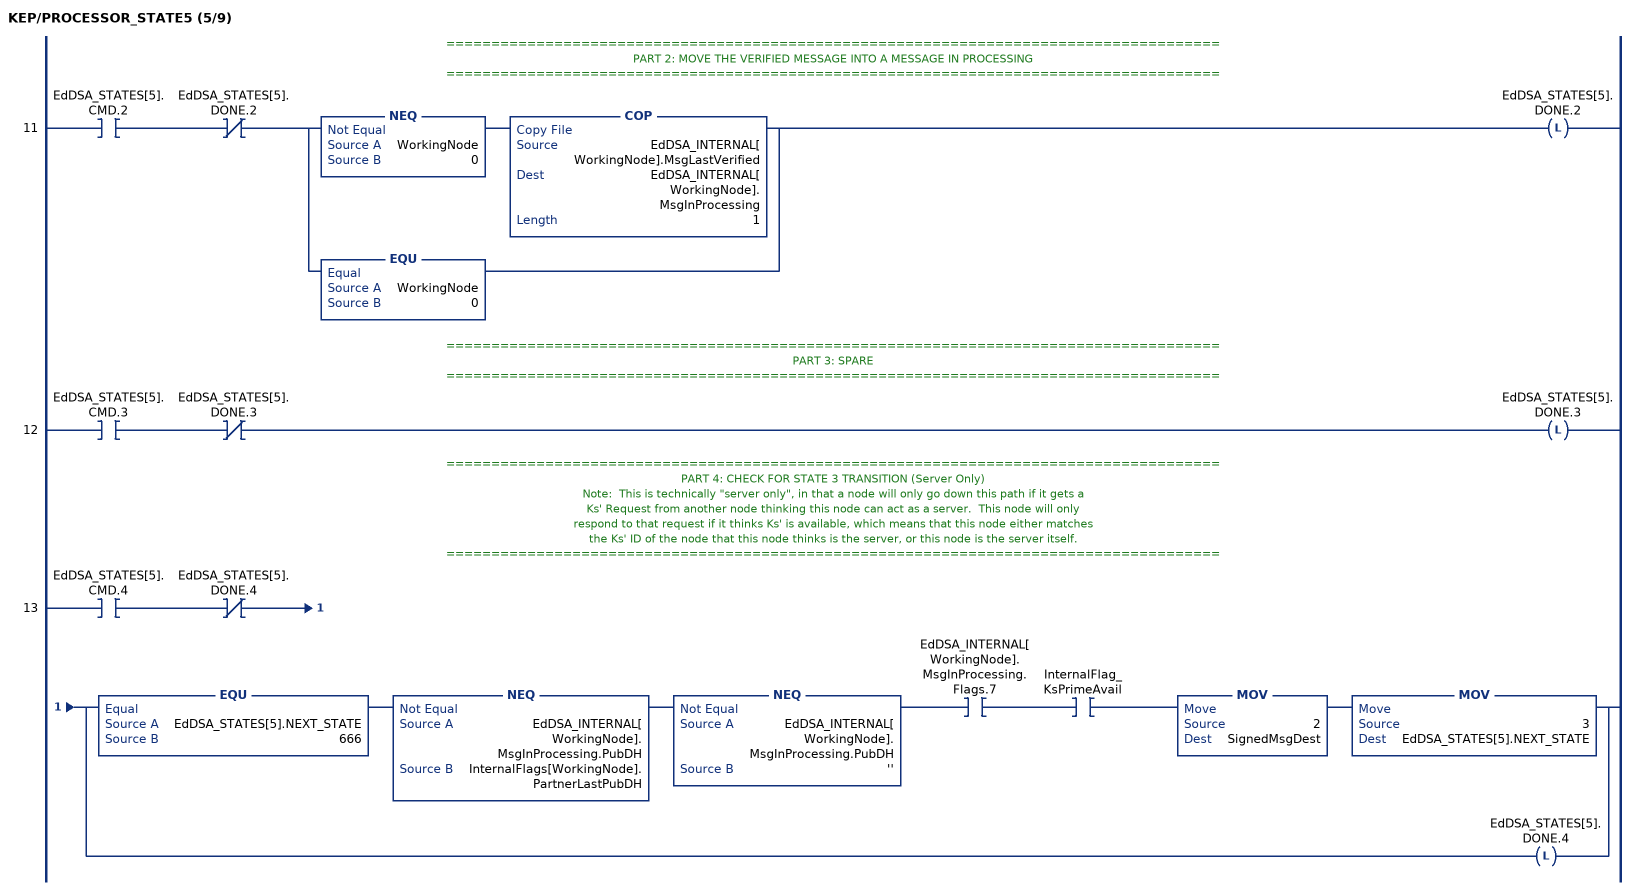
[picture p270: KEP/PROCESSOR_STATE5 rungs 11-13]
   // ======================================================================================
   // PART 2: MOVE THE VERIFIED MESSAGE INTO A MESSAGE IN PROCESSING
   // ======================================================================================
   11: XIC(EdDSA_STATES[5].CMD.2)XIO(EdDSA_STATES[5].DONE.2)[NEQ(WorkingNode,0) COP(EdDSA_INTERNAL[WorkingNode].MsgLastVerified,EdDSA_INTERNAL[WorkingNode].MsgInProcessing,1) ,EQU(WorkingNode,0) ]OTL(EdDSA_STATES[5].DONE.2);
   // ======================================================================================
   // PART 3: SPARE
   // ======================================================================================
   12: XIC(EdDSA_STATES[5].CMD.3)XIO(EdDSA_STATES[5].DONE.3)OTL(EdDSA_STATES[5].DONE.3);
   // ======================================================================================
   // PART 4: CHECK FOR STATE 3 TRANSITION (Server Only)
   // Note:  This is technically "server only", in that a node will only go down this path if it gets a
   // Ks' Request from another node thinking this node can act as a server.  This node will only
   // respond to that request if it thinks Ks' is available, which means that this node either matches
   // the Ks' ID of the node that this node thinks is the server, or this node is the server itself.
   // ======================================================================================
   13: XIC(EdDSA_STATES[5].CMD.4)XIO(EdDSA_STATES[5].DONE.4)[EQU(EdDSA_STATES[5].NEXT_STATE,666) NEQ(EdDSA_INTERNAL[WorkingNode].MsgInProcessing.PubDH,InternalFlags[WorkingNode].PartnerLastPubDH) NEQ(EdDSA_INTERNAL[WorkingNode].MsgInProcessing.PubDH,'') XIC(EdDSA_INTERNAL[WorkingNode].MsgInProcessing.Flags.7) XIC(InternalFlag_KsPrimeAvail) MOV(2,SignedMsgDest) MOV(3,EdDSA_STATES[5].NEXT_STATE) ,OTL(EdDSA_STATES[5].DONE.4) ];
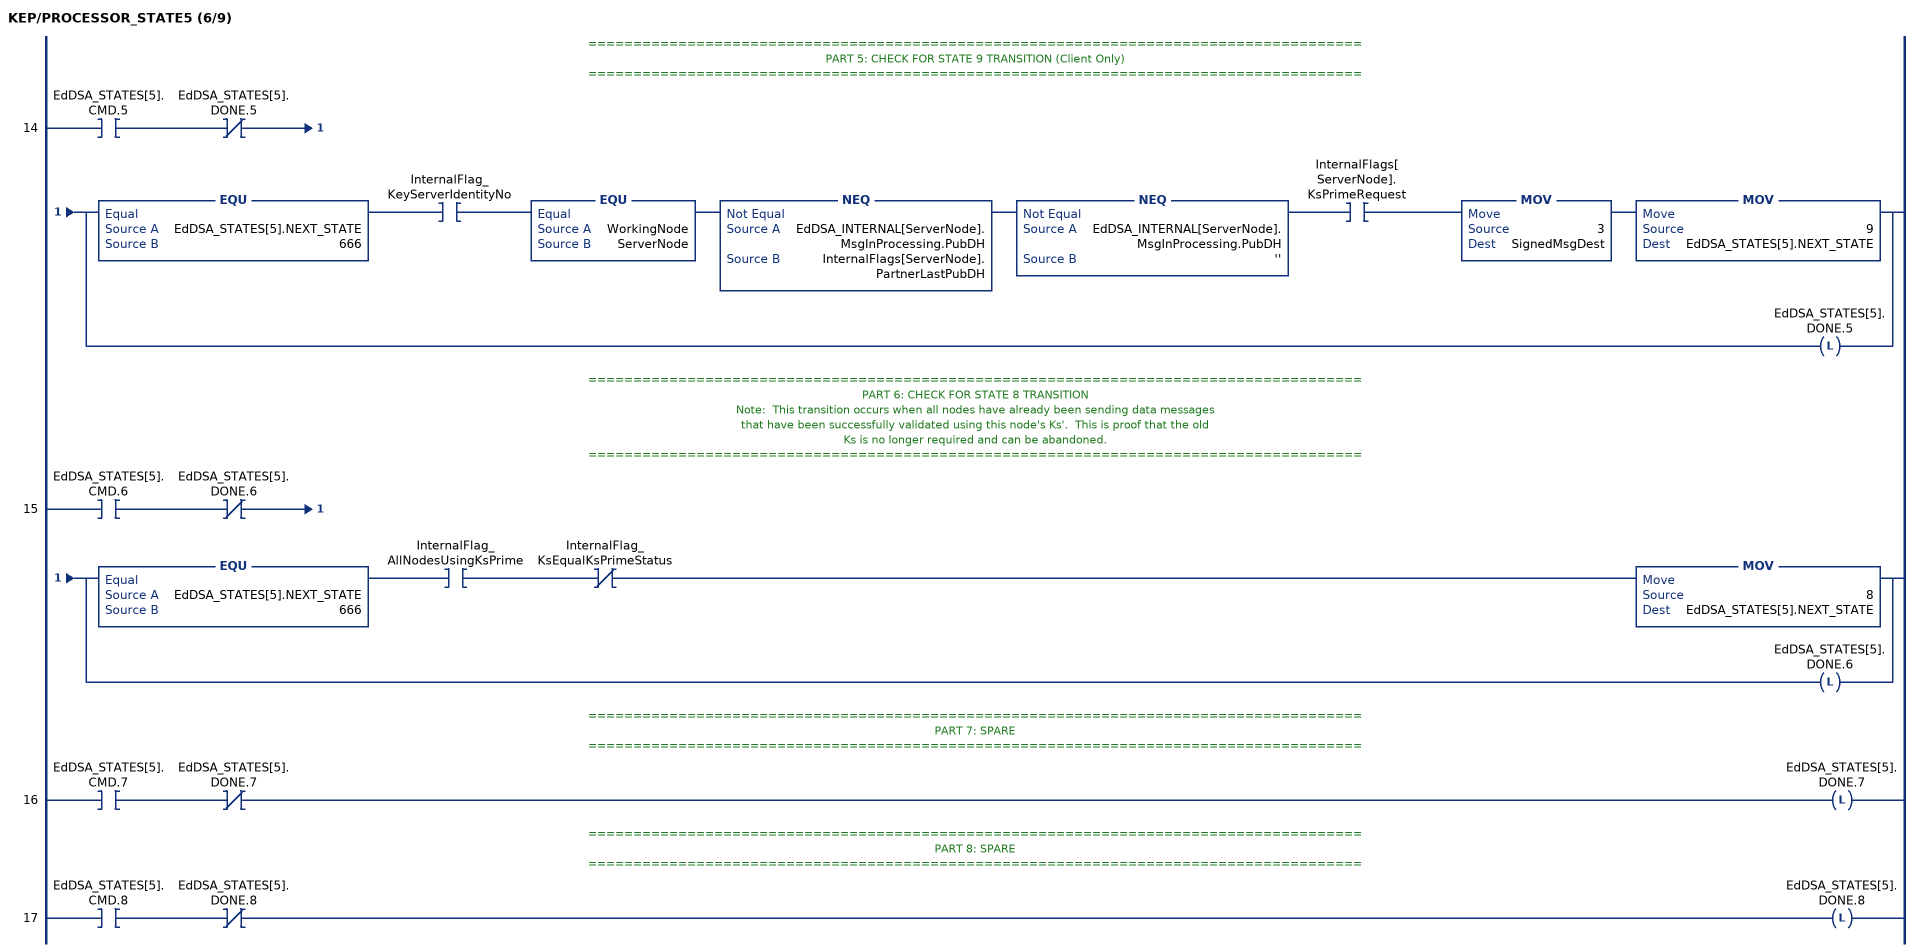
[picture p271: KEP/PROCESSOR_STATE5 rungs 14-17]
   // ======================================================================================
   // PART 5: CHECK FOR STATE 9 TRANSITION (Client Only)
   // ======================================================================================
   14: XIC(EdDSA_STATES[5].CMD.5)XIO(EdDSA_STATES[5].DONE.5)[EQU(EdDSA_STATES[5].NEXT_STATE,666) XIC(InternalFlag_KeyServerIdentityNo) EQU(WorkingNode,ServerNode) NEQ(EdDSA_INTERNAL[ServerNode].MsgInProcessing.PubDH,InternalFlags[ServerNode].PartnerLastPubDH) NEQ(EdDSA_INTERNAL[ServerNode].MsgInProcessing.PubDH,'') XIC(InternalFlags[ServerNode].KsPrimeRequest) MOV(3,SignedMsgDest) MOV(9,EdDSA_STATES[5].NEXT_STATE) ,OTL(EdDSA_STATES[5].DONE.5) ];
   // ======================================================================================
   // PART 6: CHECK FOR STATE 8 TRANSITION
   // Note:  This transition occurs when all nodes have already been sending data messages
   // that have been successfully validated using this node's Ks'.  This is proof that the old
   // Ks is no longer required and can be abandoned.
   // ======================================================================================
   15: XIC(EdDSA_STATES[5].CMD.6)XIO(EdDSA_STATES[5].DONE.6)[EQU(EdDSA_STATES[5].NEXT_STATE,666) XIC(InternalFlag_AllNodesUsingKsPrime) XIO(InternalFlag_KsEqualKsPrimeStatus) MOV(8,EdDSA_STATES[5].NEXT_STATE) ,OTL(EdDSA_STATES[5].DONE.6) ];
   // ======================================================================================
   // PART 7: SPARE
   // ======================================================================================
   16: XIC(EdDSA_STATES[5].CMD.7)XIO(EdDSA_STATES[5].DONE.7)OTL(EdDSA_STATES[5].DONE.7);
   // ======================================================================================
   // PART 8: SPARE
   // ======================================================================================
   17: XIC(EdDSA_STATES[5].CMD.8)XIO(EdDSA_STATES[5].DONE.8)OTL(EdDSA_STATES[5].DONE.8);
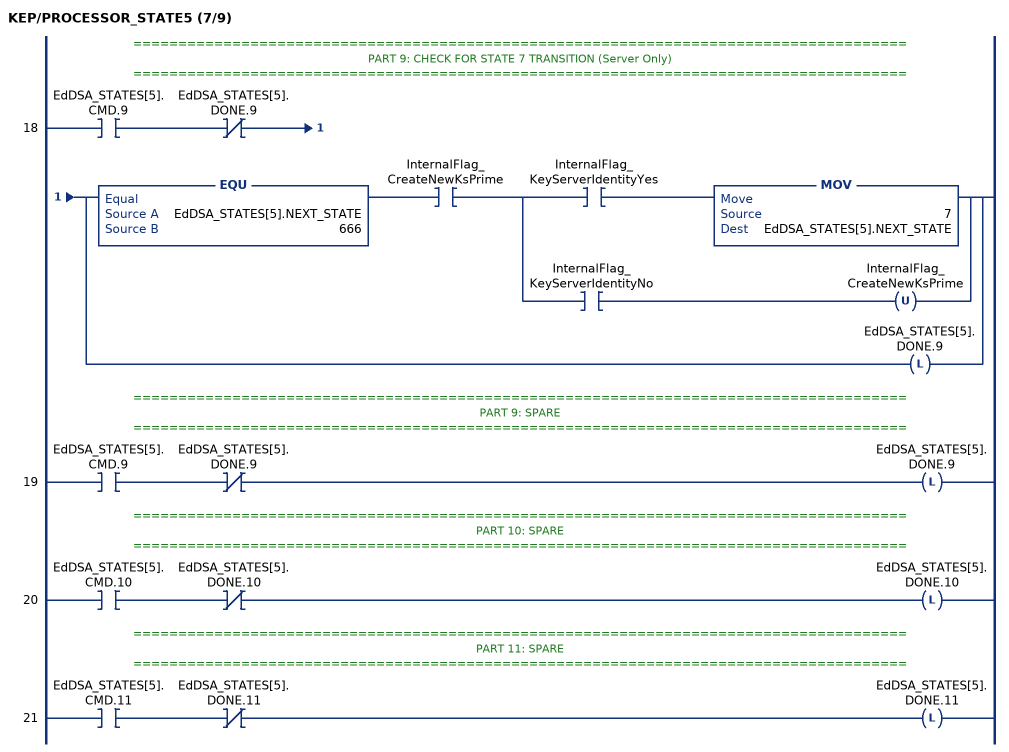
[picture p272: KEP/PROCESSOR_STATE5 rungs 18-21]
   // ======================================================================================
   // PART 9: CHECK FOR STATE 7 TRANSITION (Server Only)
   // ======================================================================================
   18: XIC(EdDSA_STATES[5].CMD.9)XIO(EdDSA_STATES[5].DONE.9)[EQU(EdDSA_STATES[5].NEXT_STATE,666) XIC(InternalFlag_CreateNewKsPrime) [XIC(InternalFlag_KeyServerIdentityYes) MOV(7,EdDSA_STATES[5].NEXT_STATE) ,XIC(InternalFlag_KeyServerIdentityNo) OTU(InternalFlag_CreateNewKsPrime) ] ,OTL(EdDSA_STATES[5].DONE.9) ];
   // ======================================================================================
   // PART 9: SPARE
   // ======================================================================================
   19: XIC(EdDSA_STATES[5].CMD.9)XIO(EdDSA_STATES[5].DONE.9)OTL(EdDSA_STATES[5].DONE.9);
   // ======================================================================================
   // PART 10: SPARE
   // ======================================================================================
   20: XIC(EdDSA_STATES[5].CMD.10)XIO(EdDSA_STATES[5].DONE.10)OTL(EdDSA_STATES[5].DONE.10);
   // ======================================================================================
   // PART 11: SPARE
   // ======================================================================================
   21: XIC(EdDSA_STATES[5].CMD.11)XIO(EdDSA_STATES[5].DONE.11)OTL(EdDSA_STATES[5].DONE.11);
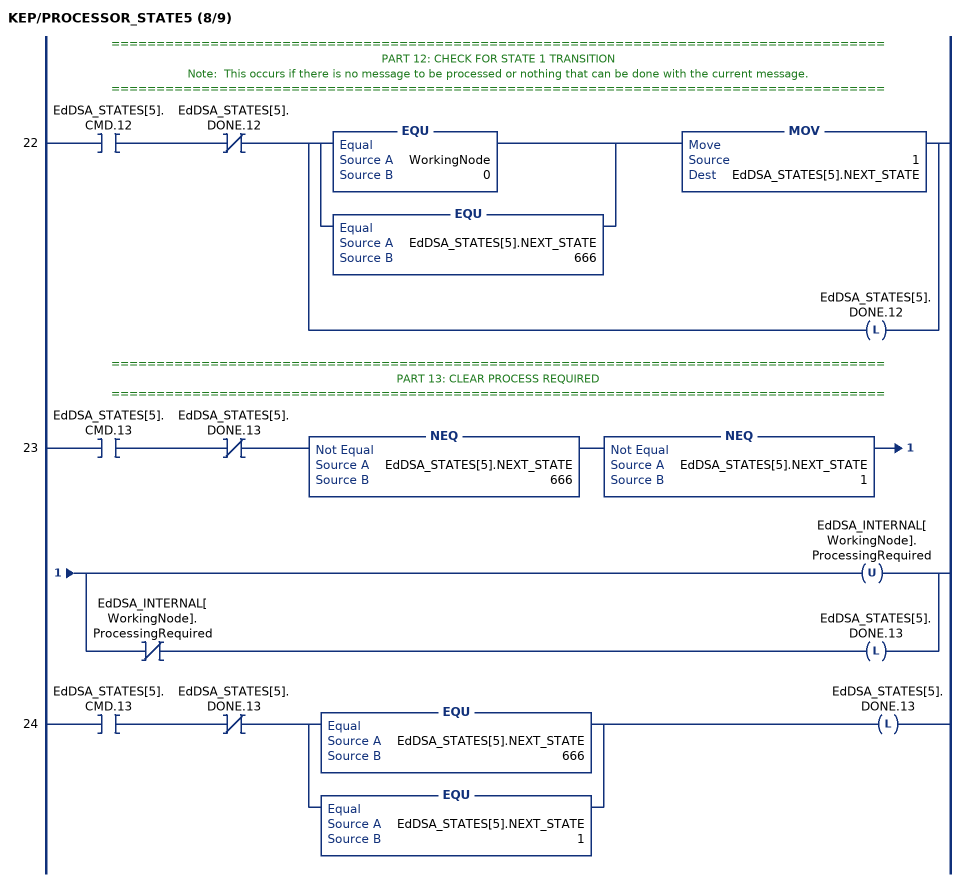
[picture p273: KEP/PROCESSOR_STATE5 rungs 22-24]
   // ======================================================================================
   // PART 12: CHECK FOR STATE 1 TRANSITION
   // Note:  This occurs if there is no message to be processed or nothing that can be done with the current message.
   // ======================================================================================
   22: XIC(EdDSA_STATES[5].CMD.12)XIO(EdDSA_STATES[5].DONE.12)[[EQU(WorkingNode,0) ,EQU(EdDSA_STATES[5].NEXT_STATE,666) ] MOV(1,EdDSA_STATES[5].NEXT_STATE) ,OTL(EdDSA_STATES[5].DONE.12) ];
   // ======================================================================================
   // PART 13: CLEAR PROCESS REQUIRED
   // ======================================================================================
   23: XIC(EdDSA_STATES[5].CMD.13)XIO(EdDSA_STATES[5].DONE.13)NEQ(EdDSA_STATES[5].NEXT_STATE,666)NEQ(EdDSA_STATES[5].NEXT_STATE,1)[OTU(EdDSA_INTERNAL[WorkingNode].ProcessingRequired) ,XIO(EdDSA_INTERNAL[WorkingNode].ProcessingRequired) OTL(EdDSA_STATES[5].DONE.13) ];
   24: XIC(EdDSA_STATES[5].CMD.13)XIO(EdDSA_STATES[5].DONE.13)[EQU(EdDSA_STATES[5].NEXT_STATE,666) ,EQU(EdDSA_STATES[5].NEXT_STATE,1) ]OTL(EdDSA_STATES[5].DONE.13);
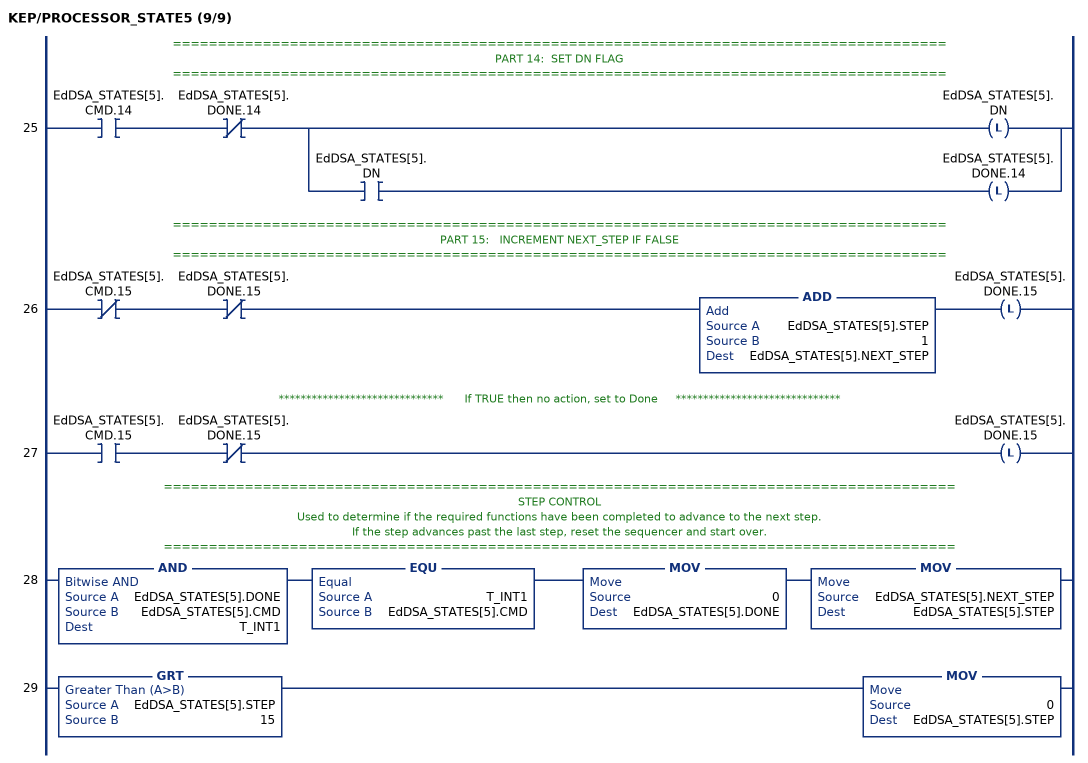
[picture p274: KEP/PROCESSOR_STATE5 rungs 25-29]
   // ======================================================================================
   // PART 14:  SET DN FLAG
   // ======================================================================================
   25: XIC(EdDSA_STATES[5].CMD.14)XIO(EdDSA_STATES[5].DONE.14)[OTL(EdDSA_STATES[5].DN) ,XIC(EdDSA_STATES[5].DN) OTL(EdDSA_STATES[5].DONE.14) ];
   // ======================================================================================
   // PART 15:   INCREMENT NEXT_STEP IF FALSE
   // ======================================================================================
   26: XIO(EdDSA_STATES[5].CMD.15)XIO(EdDSA_STATES[5].DONE.15)ADD(EdDSA_STATES[5].STEP,1,EdDSA_STATES[5].NEXT_STEP)OTL(EdDSA_STATES[5].DONE.15);
   // ******************************      If TRUE then no action, set to Done     ******************************
   27: XIC(EdDSA_STATES[5].CMD.15)XIO(EdDSA_STATES[5].DONE.15)OTL(EdDSA_STATES[5].DONE.15);
   // ========================================================================================
   // STEP CONTROL
   // Used to determine if the required functions have been completed to advance to the next step.
   // If the step advances past the last step, reset the sequencer and start over.
   // ========================================================================================
   28: AND(EdDSA_STATES[5].DONE,EdDSA_STATES[5].CMD,T_INT1)EQU(T_INT1,EdDSA_STATES[5].CMD)MOV(0,EdDSA_STATES[5].DONE)MOV(EdDSA_STATES[5].NEXT_STEP,EdDSA_STATES[5].STEP);
   29: GRT(EdDSA_STATES[5].STEP,15)MOV(0,EdDSA_STATES[5].STEP);
END_ROUTINE
